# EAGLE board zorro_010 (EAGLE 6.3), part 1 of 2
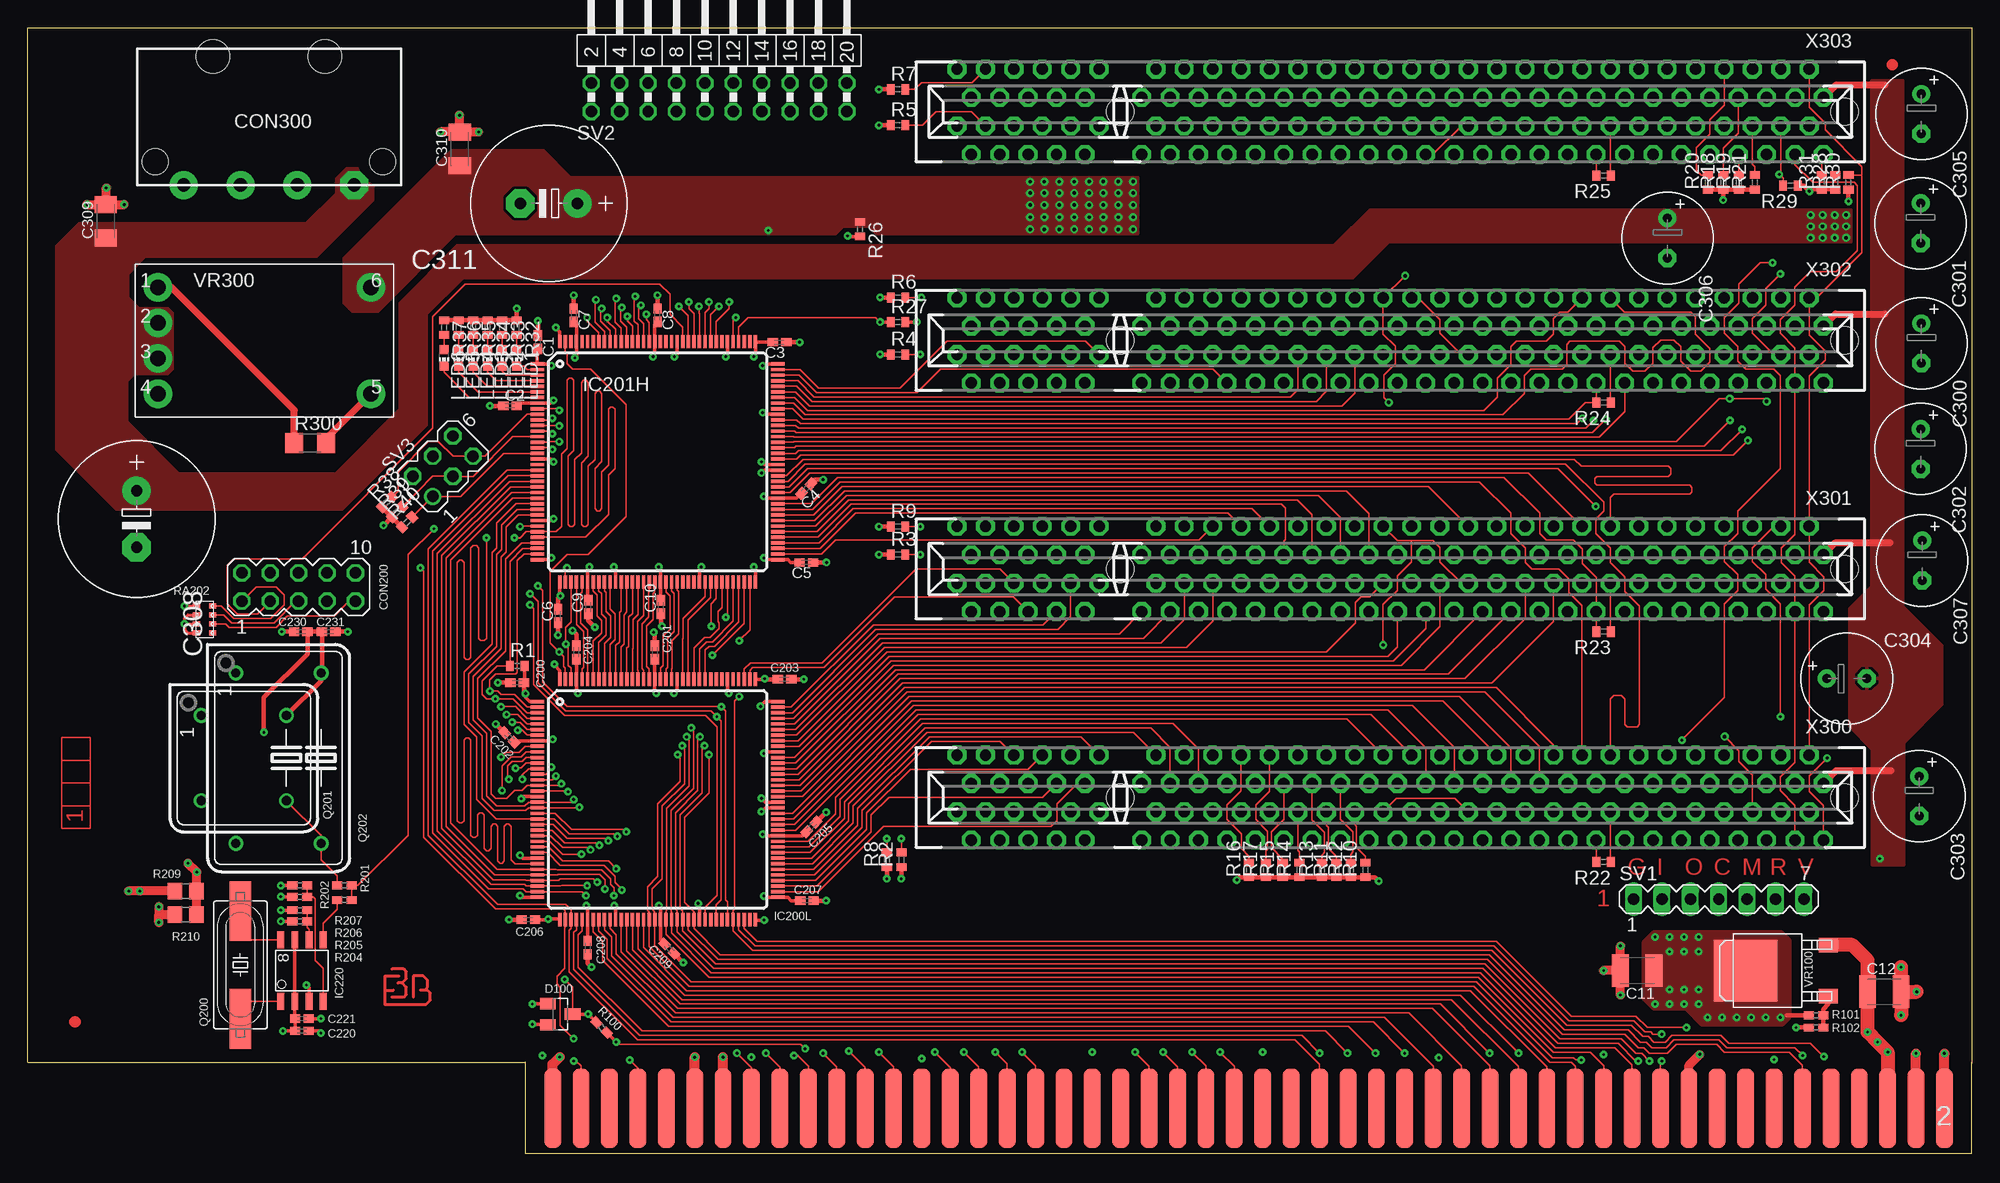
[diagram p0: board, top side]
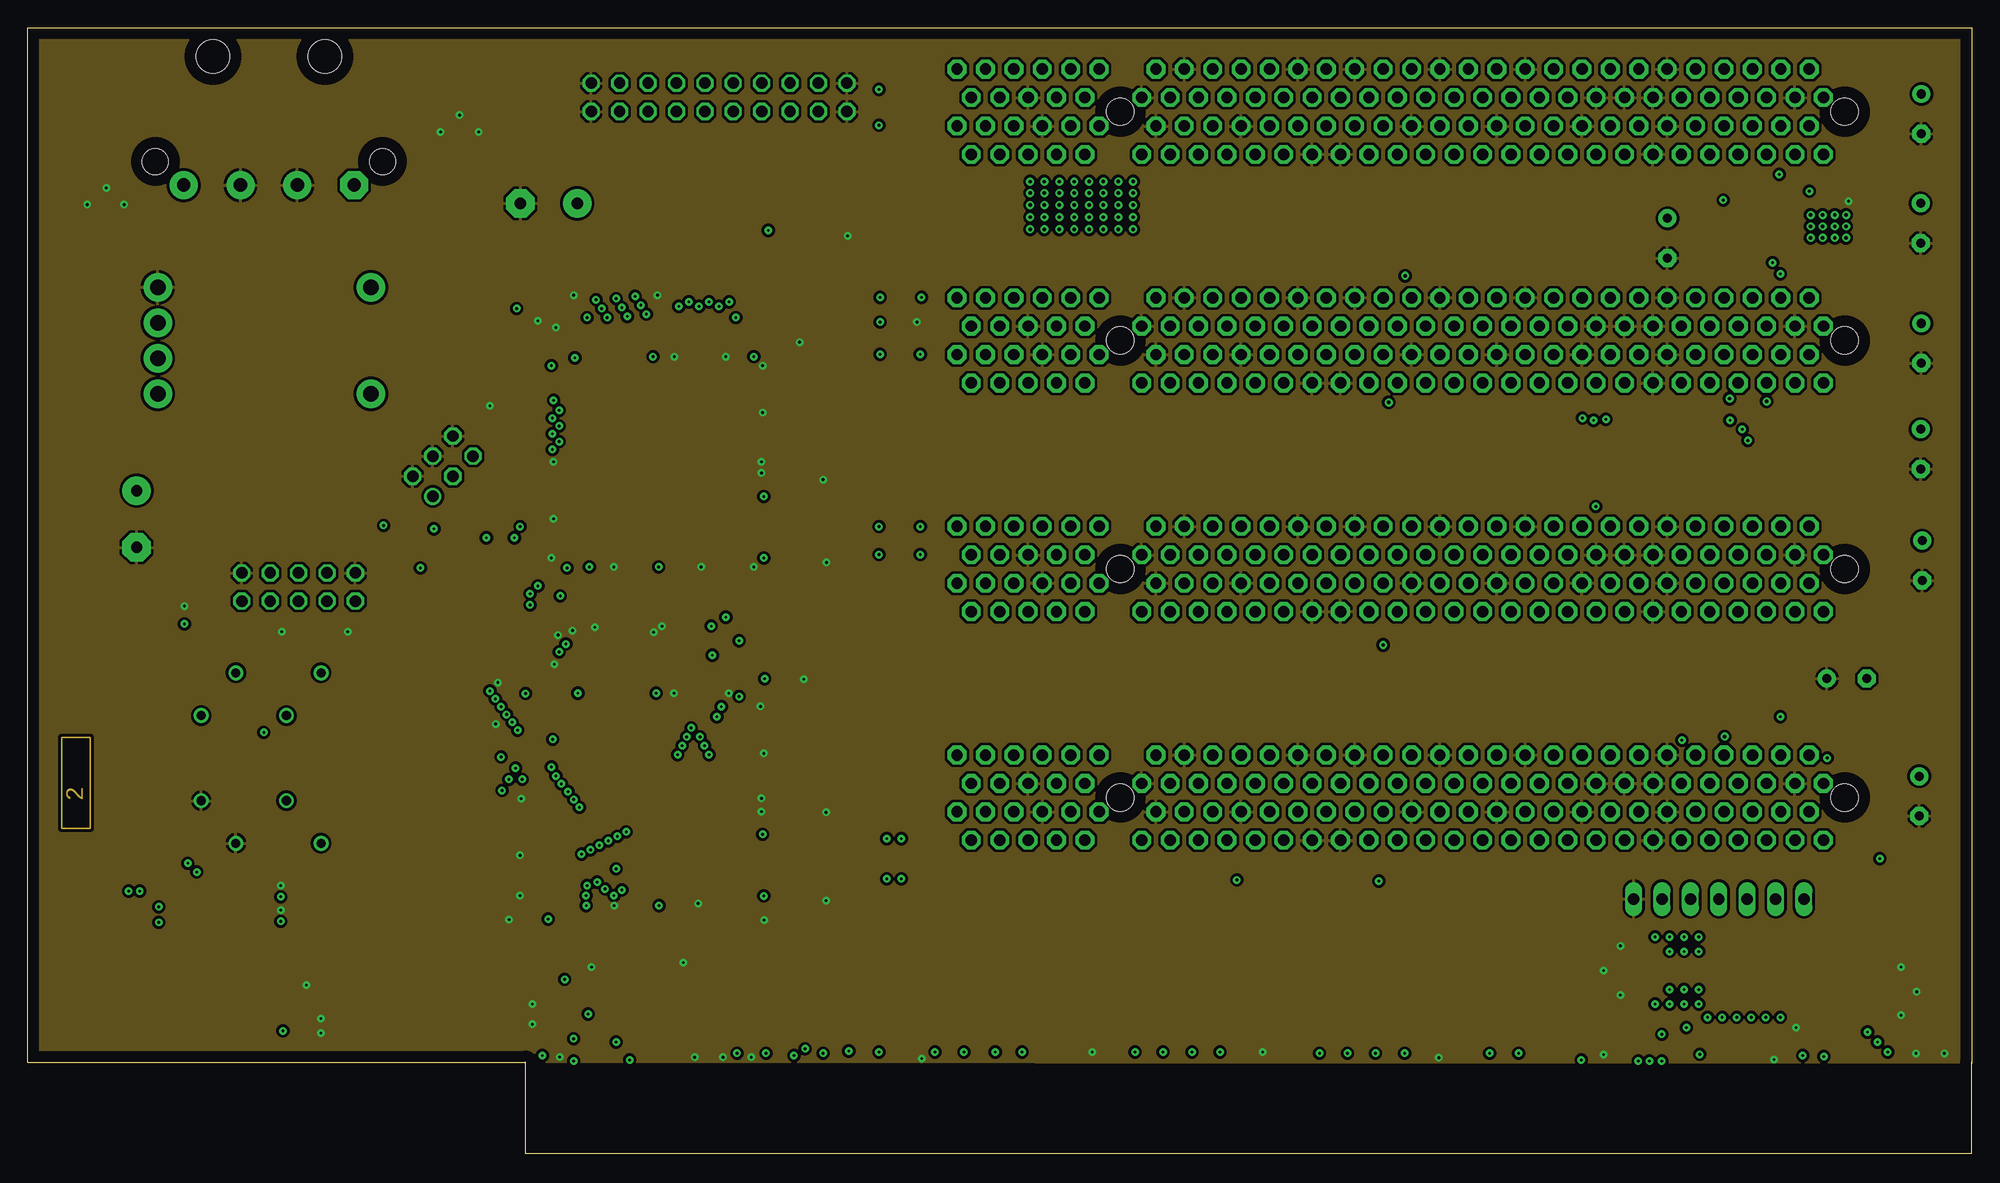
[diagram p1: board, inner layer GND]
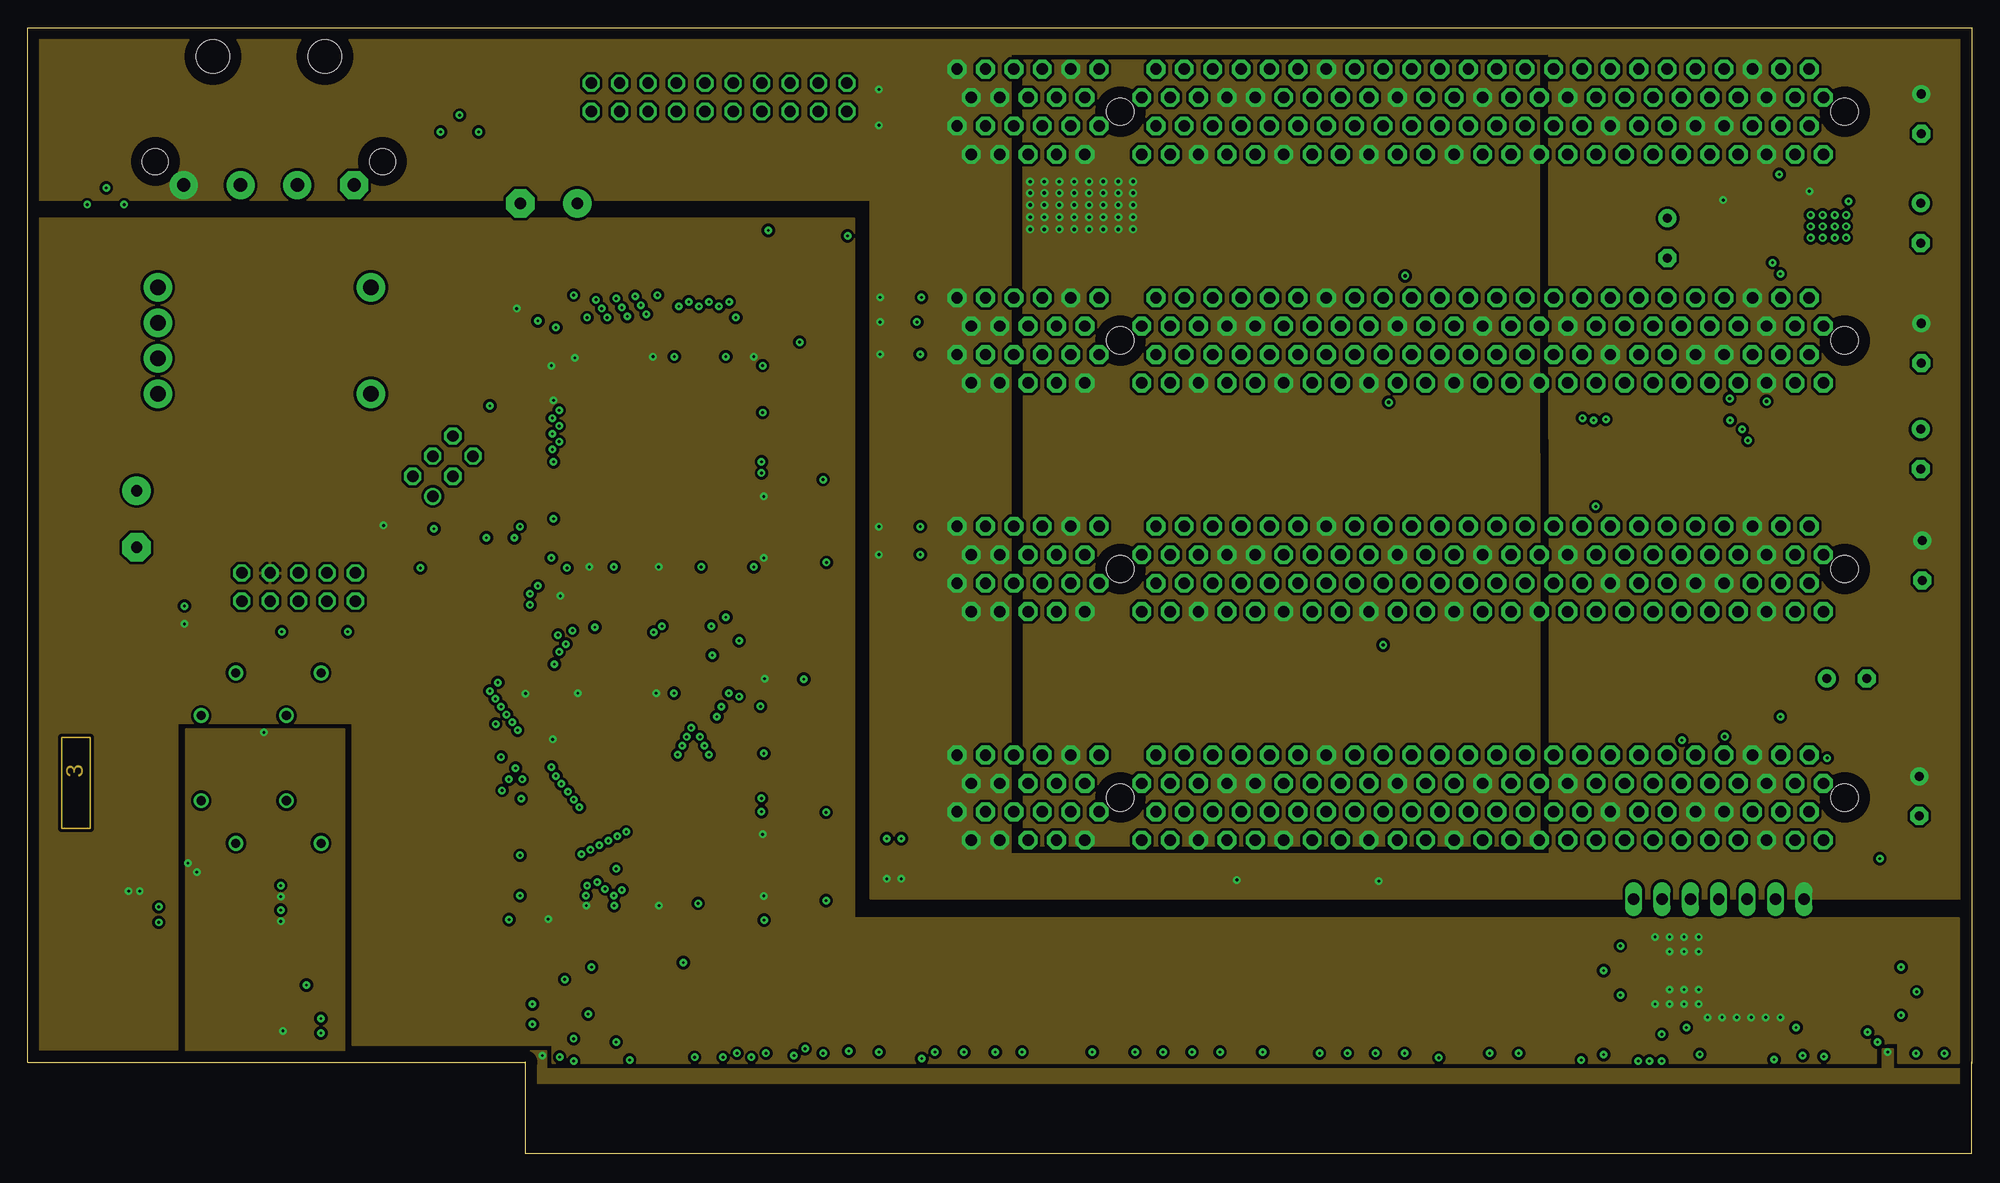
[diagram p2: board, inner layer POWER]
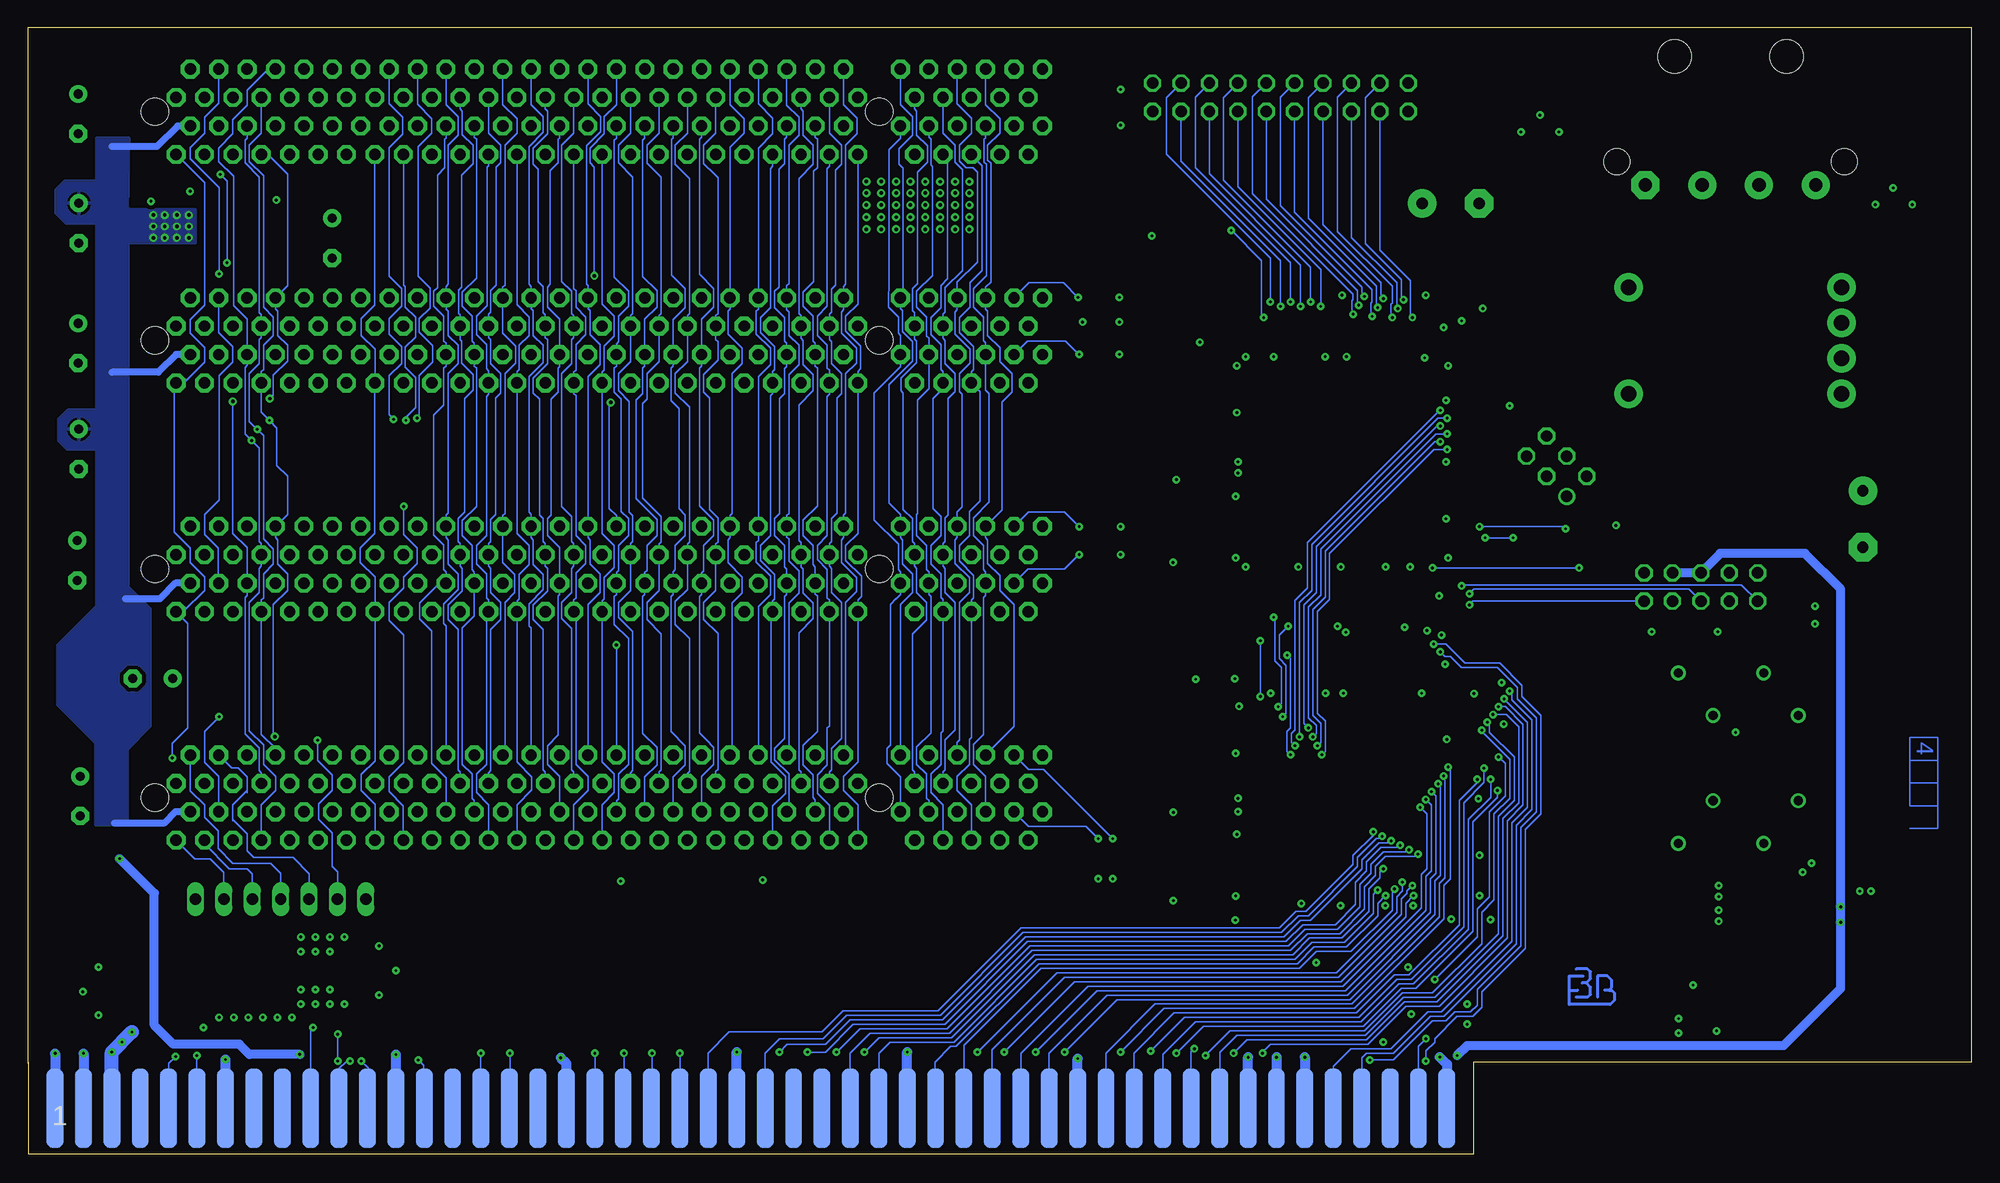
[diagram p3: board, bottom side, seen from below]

Size 173.8 x 100.67 mm. Coordinates in mm from the lower left corner, seen from the top.
Outline: 173.8,8.07 173.8,100.67 0,100.67 0,8.17 44.5,8.17
Copper layers (1+2*15+16): Top 0.035mm / dielectric 0.2mm / GND 0.035mm / dielectric 1.5mm / POWER 0.035mm / dielectric 0.2mm / Bottom 0.035mm
Design rules "default": minimum track width 6mil, minimum drill 8mil, track to track 6mil, track to pad 6mil, pad to pad 6mil, via to via 6mil, smd to smd 6mil, copper to edge 40mil, drill to drill 12mil, minimum pad ring 10mil, minimum via ring 8mil, stop-mask expansion 0mil, vias tented up to drill 0mil, thermal gap 10mil

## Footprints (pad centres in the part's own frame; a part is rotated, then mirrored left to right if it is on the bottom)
C0402K = smd 0.925 x 0.74: 1 -0.6,0; 2 0.6,0
C1210K = smd 1.5 x 2.9: 1 -1.5,0; 2 1.5,0
E3,5-8 = drill 0.813 pad 1.6: + -1.778,0 | drill 0.813 pad 1.6 octagon: - 1.778,0
E5-13 = drill 1.016 pad 2.54: + -2.54,0 | drill 1.016 pad 2.54 octagon: - 2.54,0
C1206K = smd 1.5 x 2: 1 -1.5,0; 2 1.5,0
ZORROM = smd 1.524 x 7.096 bottom: 1 0,4.08; 3 -2.54,4.08; 5 -5.08,4.08; 7 -7.62,4.08; 9 -10.16,4.08; 11 -12.7,4.08; 13 -15.24,4.08; 15 -17.78,4.08; 17 -20.32,4.08; 19 -22.86,4.08; 21 -25.4,4.08; 23 -27.94,4.08; 25 -30.48,4.08; 27 -33.02,4.08; 29 -35.56,4.08; 31 -38.1,4.08; 33 -40.64,4.08; 35 -43.18,4.08; 37 -45.72,4.08; 39 -48.26,4.08; 41 -50.8,4.08; 43 -53.34,4.08; 45 -55.88,4.08; 47 -58.42,4.08; 49 -60.96,4.08; 51 -63.5,4.08; 53 -66.04,4.08; 55 -68.58,4.08; 57 -71.12,4.08; 59 -73.66,4.08; 61 -76.2,4.08; 63 -78.74,4.08; 65 -81.28,4.08; 67 -83.82,4.08; 69 -86.36,4.08; 71 -88.9,4.08; 73 -91.44,4.08; 75 -93.98,4.08; 77 -96.52,4.08; 79 -99.06,4.08; 81 -101.6,4.08; 83 -104.14,4.08; 85 -106.68,4.08; 87 -109.22,4.08; 89 -111.76,4.08; 91 -114.3,4.08; 93 -116.84,4.08; 95 -119.38,4.08; 97 -121.92,4.08; 99 -124.46,4.08 | smd 1.524 x 7.096: 2 0,4.08; 4 -2.54,4.08; 6 -5.08,4.08; 8 -7.62,4.08; 10 -10.16,4.08; 12 -12.7,4.08; 14 -15.24,4.08; 16 -17.78,4.08; 18 -20.32,4.08; 20 -22.86,4.08; 22 -25.4,4.08; 24 -27.94,4.08; 26 -30.48,4.08; 28 -33.02,4.08; 30 -35.56,4.08; 32 -38.1,4.08; 34 -40.64,4.08; 36 -43.18,4.08; 38 -45.72,4.08; 40 -48.26,4.08; 42 -50.8,4.08; 44 -53.34,4.08; 46 -55.88,4.08; 48 -58.42,4.08; 50 -60.96,4.08; 52 -63.5,4.08; 54 -66.04,4.08; 56 -68.58,4.08; 58 -71.12,4.08; 60 -73.66,4.08; 62 -76.2,4.08; 64 -78.74,4.08; 66 -81.28,4.08; 68 -83.82,4.08; 70 -86.36,4.08; 72 -88.9,4.08; 74 -91.44,4.08; 76 -93.98,4.08; 78 -96.52,4.08; 80 -99.06,4.08; 82 -101.6,4.08; 84 -104.14,4.08; 86 -106.68,4.08; 88 -109.22,4.08; 90 -111.76,4.08; 92 -114.3,4.08; 94 -116.84,4.08; 96 -119.38,4.08; 98 -121.92,4.08; 100 -124.46,4.08
MA05-2 = drill 1.016 octagon: 1 -5.08,-1.27; 2 -5.08,1.27; 3 -2.54,-1.27; 4 -2.54,1.27; 5 0,-1.27; 6 0,1.27; 7 2.54,-1.27; 8 2.54,1.27; 9 5.08,-1.27; 10 5.08,1.27
5.25A = drill 1.2 pad 2.5 octagon: 1 -7.62,0 | drill 1.2 pad 2.5: 2 -2.54,0; 3 2.54,0; 4 7.62,0 | hole 2.3: -10.16,-2.1; 10.16,-2.1 | hole 3: -5,-11.5; 5,-11.5
SOT23 = smd 1 x 1.4: 1 -0.95,-1.1; 2 0.95,-1.1; 3 0,1.1
TQFP144 = smd 1.2 x 0.3: 1 -10.75,8.75; 2 -10.75,8.25; 3 -10.75,7.75; 4 -10.75,7.25; 5 -10.75,6.75; 6 -10.75,6.25; 7 -10.75,5.75; 8 -10.75,5.25; 9 -10.75,4.75; 10 -10.75,4.25; 11 -10.75,3.75; 12 -10.75,3.25; 13 -10.75,2.75; 14 -10.75,2.25; 15 -10.75,1.75; 16 -10.75,1.25; 17 -10.75,0.75; 18 -10.75,0.25; 19 -10.75,-0.25; 20 -10.75,-0.75; 21 -10.75,-1.25; 22 -10.75,-1.75; 23 -10.75,-2.25; 24 -10.75,-2.75; 25 -10.75,-3.25; 26 -10.75,-3.75; 27 -10.75,-4.25; 28 -10.75,-4.75; 29 -10.75,-5.25; 30 -10.75,-5.75; 31 -10.75,-6.25; 32 -10.75,-6.75; 33 -10.75,-7.25; 34 -10.75,-7.75; 35 -10.75,-8.25; 36 -10.75,-8.75; 73 10.75,-8.75; 74 10.75,-8.25; 75 10.75,-7.75; 76 10.75,-7.25; 77 10.75,-6.75; 78 10.75,-6.25; 79 10.75,-5.75; 80 10.75,-5.25; 81 10.75,-4.75; 82 10.75,-4.25; 83 10.75,-3.75; 84 10.75,-3.25; 85 10.75,-2.75; 86 10.75,-2.25; 87 10.75,-1.75; 88 10.75,-1.25; 89 10.75,-0.75; 90 10.75,-0.25; 91 10.75,0.25; 92 10.75,0.75; 93 10.75,1.25; 94 10.75,1.75; 95 10.75,2.25; 96 10.75,2.75; 97 10.75,3.25; 98 10.75,3.75; 99 10.75,4.25; 100 10.75,4.75; 101 10.75,5.25; 102 10.75,5.75; 103 10.75,6.25; 104 10.75,6.75; 105 10.75,7.25; 106 10.75,7.75; 107 10.75,8.25; 108 10.75,8.75 | smd 0.3 x 1.2: 37 -8.75,-10.75; 38 -8.25,-10.75; 39 -7.75,-10.75; 40 -7.25,-10.75; 41 -6.75,-10.75; 42 -6.25,-10.75; 43 -5.75,-10.75; 44 -5.25,-10.75; 45 -4.75,-10.75; 46 -4.25,-10.75; 47 -3.75,-10.75; 48 -3.25,-10.75; 49 -2.75,-10.75; 50 -2.25,-10.75; 51 -1.75,-10.75; 52 -1.25,-10.75; 53 -0.75,-10.75; 54 -0.25,-10.75; 55 0.25,-10.75; 56 0.75,-10.75; 57 1.25,-10.75; 58 1.75,-10.75; 59 2.25,-10.75; 60 2.75,-10.75; 61 3.25,-10.75; 62 3.75,-10.75; 63 4.25,-10.75; 64 4.75,-10.75; 65 5.25,-10.75; 66 5.75,-10.75; 67 6.25,-10.75; 68 6.75,-10.75; 69 7.25,-10.75; 70 7.75,-10.75; 71 8.25,-10.75; 72 8.75,-10.75; 109 8.75,10.75; 110 8.25,10.75; 111 7.75,10.75; 112 7.25,10.75; 113 6.75,10.75; 114 6.25,10.75; 115 5.75,10.75; 116 5.25,10.75; 117 4.75,10.75; 118 4.25,10.75; 119 3.75,10.75; 120 3.25,10.75; 121 2.75,10.75; 122 2.25,10.75; 123 1.75,10.75; 124 1.25,10.75; 125 0.75,10.75; 126 0.25,10.75; 127 -0.25,10.75; 128 -0.75,10.75; 129 -1.25,10.75; 130 -1.75,10.75; 131 -2.25,10.75; 132 -2.75,10.75; 133 -3.25,10.75; 134 -3.75,10.75; 135 -4.25,10.75; 136 -4.75,10.75; 137 -5.25,10.75; 138 -5.75,10.75; 139 -6.25,10.75; 140 -6.75,10.75; 141 -7.25,10.75; 142 -7.75,10.75; 143 -8.25,10.75; 144 -8.75,10.75
SO8 = smd 0.61 x 1.524: 1 -1.905,-2.743; 2 -0.635,-2.743; 3 0.635,-2.743; 4 1.905,-2.743; 5 1.905,2.743; 6 0.635,2.743; 7 -0.635,2.743; 8 -1.905,2.743
CHIP-LED0603 = smd 0.8 x 0.8: A 0,-0.75; C 0,0.75
HC49UP = smd 5.334 x 1.93: 1 -4.826,0; 2 4.826,0
DIL08S = drill 0.813: 1 -3.81,-3.81; 4 3.81,-3.81; 5 3.81,3.81; 8 -3.81,3.81
DIL14S = drill 0.813: 1 -7.62,-3.81; 7 7.62,-3.81; 8 7.62,3.81; 14 -7.62,3.81
R0402 = smd 0.7 x 0.9: 1 -0.65,0; 2 0.65,0
R0402@1 = smd 0.9 x 0.7: 1 -0.65,0; 2 0.65,0
R0805@1 = smd 1.3 x 1.5: 1 -0.95,0; 2 0.95,0
R1206 = smd 1.6 x 1.803: 1 -1.422,0; 2 1.422,0
RARRAY4 = smd 0.45 x 0.65: 1 -1.2,-0.725; 2 -0.4,-0.725; 3 0.4,-0.725; 4 1.2,-0.725; 5 1.2,0.725; 6 0.4,0.725; 7 -0.4,0.725; 8 -1.2,0.725
MA07-1 = drill 1.016 long: 1 -7.62,0; 2 -5.08,0; 3 -2.54,0; 4 0,0; 5 2.54,0; 6 5.08,0; 7 7.62,0
MA10-2W = drill 1.016 octagon: 1 -11.43,-1.27; 2 -11.43,1.27; 3 -8.89,-1.27; 4 -8.89,1.27; 5 -6.35,-1.27; 6 -6.35,1.27; 7 -3.81,-1.27; 8 -3.81,1.27; 9 -1.27,-1.27; 10 -1.27,1.27; 11 1.27,-1.27; 12 1.27,1.27; 13 3.81,-1.27; 14 3.81,1.27; 15 6.35,-1.27; 16 6.35,1.27; 17 8.89,-1.27; 18 8.89,1.27; 19 11.43,-1.27; 20 11.43,1.27
MA03-2 = drill 1.016: 1 -2.54,-1.27 | drill 1.016 octagon: 2 -2.54,1.27; 3 0,-1.27; 4 0,1.27; 5 2.54,-1.27; 6 2.54,1.27
TO252 = smd 1.3 x 1.7: 1 -2.285,-7.4; 3 2.285,-7.4 | smd 5.5 x 5.7: 2 0,0
PME_TH = drill 1.397 pad 2.54: 1 -9.525,4.763; 2 -9.525,1.587; 3 -9.525,-1.587; 4 -9.525,-4.763; 5 9.525,-4.763; 6 9.525,4.763
CON-PCI = drill 1.016 pad 1.676 octagon: A1 -38.735,3.81; A2 -37.465,1.27; A3 -36.195,3.81; A4 -34.925,1.27; A5 -33.655,3.81; A6 -32.385,1.27; A7 -31.115,3.81; A8 -29.845,1.27; A9 -28.575,3.81; A10 -27.305,1.27; A11 -26.035,3.81; A12 -24.765,1.27; A13 -23.495,3.81; A14 -22.225,1.27; A15 -20.955,3.81; A16 -19.685,1.27; A17 -18.415,3.81; A18 -17.145,1.27; A19 -15.875,3.81; A20 -14.605,1.27; A21 -13.335,3.81; A22 -12.065,1.27; A23 -10.795,3.81; A24 -9.525,1.27; A25 -8.255,3.81; A26 -6.985,1.27; A27 -5.715,3.81; A28 -4.445,1.27; A29 -3.175,3.81; A30 -1.905,1.27; A31 -0.635,3.81; A32 0.635,1.27; A33 1.905,3.81; A34 3.175,1.27; A35 4.445,3.81; A36 5.715,1.27; A37 6.985,3.81; A38 8.255,1.27; A39 9.525,3.81; A40 10.795,1.27; A41 12.065,3.81; A42 13.335,1.27; A43 14.605,3.81; A44 15.875,1.27; A45 17.145,3.81; A46 18.415,1.27; A47 19.685,3.81; A48 20.955,1.27; A49 22.225,3.81; A52 26.035,1.27; A53 27.305,3.81; A54 28.575,1.27; A55 29.845,3.81; A56 31.115,1.27; A57 32.385,3.81; A58 33.655,1.27; A59 34.925,3.81; A60 36.195,1.27; A61 37.465,3.81; A62 38.735,1.27; B1 -38.735,-1.27; B2 -37.465,-3.81; B3 -36.195,-1.27; B4 -34.925,-3.81; B5 -33.655,-1.27; B6 -32.385,-3.81; B7 -31.115,-1.27; B8 -29.845,-3.81; B9 -28.575,-1.27; B10 -27.305,-3.81; B11 -26.035,-1.27; B12 -24.765,-3.81; B13 -23.495,-1.27; B14 -22.225,-3.81; B15 -20.955,-1.27; B16 -19.685,-3.81; B17 -18.415,-1.27; B18 -17.145,-3.81; B19 -15.875,-1.27; B20 -14.605,-3.81; B21 -13.335,-1.27; B22 -12.065,-3.81; B23 -10.795,-1.27; B24 -9.525,-3.81; B25 -8.255,-1.27; B26 -6.985,-3.81; B27 -5.715,-1.27; B28 -4.445,-3.81; B29 -3.175,-1.27; B30 -1.905,-3.81; B31 -0.635,-1.27; B32 0.635,-3.81; B33 1.905,-1.27; B34 3.175,-3.81; B35 4.445,-1.27; B36 5.715,-3.81; B37 6.985,-1.27; B38 8.255,-3.81; B39 9.525,-1.27; B40 10.795,-3.81; B41 12.065,-1.27; B42 13.335,-3.81; B43 14.605,-1.27; B44 15.875,-3.81; B45 17.145,-1.27; B46 18.415,-3.81; B47 19.685,-1.27; B48 20.955,-3.81; B49 22.225,-1.27; B52 26.035,-3.81; B53 27.305,-1.27; B54 28.575,-3.81; B55 29.845,-1.27; B56 31.115,-3.81; B57 32.385,-1.27; B58 33.655,-3.81; B59 34.925,-1.27; B60 36.195,-3.81; B61 37.465,-1.27; B62 38.735,-3.81 | hole 2.438: 24.13,0; -40.64,0

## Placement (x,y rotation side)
C1  100n  [C0402K]  45.6,72.57 270 top
C2  100n  [C0402K]  43.1,66.87 0 top
C3  100n  [C0402K]  67.2,72.57 180 top
C4  100n  [C0402K]  69.6,59.47 225 top
C5  100n  [C0402K]  69.6,52.87 180 top
C6  100n  [C0402K]  47.4,48.07 90 top
C7  100n  [C0402K]  48.8,74.97 270 top
C8  100n  [C0402K]  56.3,74.97 270 top
C9  100n  [C0402K]  50.1,48.87 90 top
C10  100n  [C0402K]  56.6,48.87 90 top
C11  [C1210K]  143.9,16.37 180 top
C12  [C1210K]  166,14.47 0 top
C200  100n  [C0402K]  43.75,42.12 0 top
C201  100n  [C0402K]  56.05,44.82 270 top
C202  100n  [C0402K]  43.05,37.22 315 top
C203  100n  [C0402K]  67.65,42.42 180 top
C204  100n  [C0402K]  49.05,44.82 270 top
C205  100n  [C0402K]  70.05,29.22 225 top
C206  100n  [C0402K]  44.75,20.92 0 top
C207  100n  [C0402K]  69.65,22.62 180 top
C208  100n  [C0402K]  50.05,18.42 90 top
C209  100n  [C0402K]  57.35,18.32 135 top
C220  DNU  [C0402K]  24.5,10.97 180 top
C221  DNU  [C0402K]  24.5,12.07 180 top
C230  100n  [C0402K]  24.4,46.67 0 top
C231  10n  [C0402K]  26.9,46.67 180 top
C300  [E3,5-8]  169.32,72.48 270 top
C301  [E3,5-8]  169.25,83.21 270 top
C302  [E3,5-8]  169.25,63.02 270 top
C303  [E3,5-8]  169.13,31.96 270 top
C304  [E3,5-8]  162.65,42.48 0 top
C305  [E3,5-8]  169.32,92.99 270 top
C306  [E3,5-8]  146.61,81.87 270 top
C307  [E3,5-8]  169.38,53.05 270 top
C308  [E5-13]  9.72,56.75 270 top
C309  [C1206K]  6.95,83.38 90 top
C310  [C1206K]  38.61,89.84 90 top
C311  [E5-13]  46.58,84.98 180 top
CON100  ZORRO3MEDIUM  [ZORROM]  171.38,-0.03 0 top
CON200  DNU  [MA05-2]  24.2,50.67 0 top
CON300  [5.25A]  21.55,86.62 180 top
D100  BAT54C  [SOT23]  47.6,12.47 270 top
FID100  FIDUCIALJENS  [FID_JENS]  4.2,11.77 0 top
FID101  FIDUCIALJENS  [FID_JENS]  166.7,97.37 0 top
IC200L  XC95144XL  [TQFP144]  56.3,31.67 0 top
IC201H  XC95144XL  [TQFP144]  56.3,61.87 0 top
IC220  DNU  [SO8]  24.5,16.37 0 top
LED1  [CHIP-LED0603]  43.7,71.17 180 top
LED2  [CHIP-LED0603]  42.4,71.17 180 top
LED3  [CHIP-LED0603]  41.1,71.17 180 top
LED4  [CHIP-LED0603]  39.8,71.17 180 top
LED5  [CHIP-LED0603]  38.5,71.17 180 top
LED6  [CHIP-LED0603]  37.2,71.17 180 top
Q200  DNU  [HC49UP]  19,16.87 90 top
Q201  [DIL08S]  19.3,35.37 270 top
Q202  [DIL14S]  22.4,35.37 270 top
R1  DNU  [R0402]  43.75,43.62 0 top
R2  1k0  [R0402]  78.1,26.27 90 top
R3  1k0  [R0402]  77.8,53.57 0 top
R4  1j0  [R0402]  77.8,71.47 0 top
R5  1k0  [R0402]  77.8,91.97 0 top
R6  1j0  [R0402]  77.8,76.57 0 top
R7  1j0  [R0402]  77.8,95.17 0 top
R8  1j0  [R0402]  76.8,26.27 90 top
R9  1j0  [R0402]  77.8,56.07 0 top
R10  1j0  [R0402]  119.6,25.37 90 top
R11  1j0  [R0402]  117,25.37 90 top
R12  1j0  [R0402]  118.3,25.37 90 top
R13  1j0  [R0402]  115.7,25.37 90 top
R14  1j0  [R0402]  113.7,25.37 90 top
R15  1j0  [R0402]  112.2,25.37 90 top
R16  1j0  [R0402]  109.2,25.37 90 top
R17  1j0  [R0402]  110.7,25.37 90 top
R18  1j0  [R0402]  151.6,86.87 90 top
R19  1j0  [R0402]  153,86.87 90 top
R20  1j0  [R0402]  150.2,86.87 90 top
R21  1j0  [R0402]  154.4,86.87 90 top
R22  1j0  [R0402]  140.9,26.07 180 top
R23  1j0  [R0402]  140.9,46.67 180 top
R24  1j0  [R0402]  140.9,67.17 180 top
R25  1j0  [R0402]  140.9,87.47 180 top
R26  3k3  [R0402]  74.4,82.67 270 top
R27  4k7  [R0402]  77.8,74.37 0 top
R28  1j0  [R0402]  161.6,86.87 90 top
R29  1j0  [R0402]  157.6,86.57 180 top
R30  1j0  [R0402]  162.8,86.87 90 top
R31  1j0  [R0402]  160.4,86.87 90 top
R32  3k3  [R0402]  43.7,73.87 270 top
R33  4k7  [R0402]  42.4,73.87 270 top
R34  3k3  [R0402]  41.1,73.87 270 top
R35  4k7  [R0402]  39.8,73.87 270 top
R36  3k3  [R0402]  38.5,73.87 270 top
R37  4k7  [R0402]  37.2,73.87 270 top
R38  4k7  [R0402]  32.1,58.27 45 top
R39  3k3  [R0402]  33,57.37 45 top
R40  4k7  [R0402]  33.9,56.47 45 top
R100  15R0  [R0402@1]  51.3,11.27 135 top
R101  150R0  [R0402@1]  159.9,12.37 180 top
R102  240R0  [R0402@1]  159.9,11.27 0 top
R201  15R0  [R0402@1]  28.3,23.97 0 top
R202  DNU  [R0402@1]  28.3,22.67 0 top
R204  DNU  [R0402@1]  24.3,20.77 180 top
R205  DNU  [R0402@1]  24.3,22.97 180 top
R206  DNU  [R0402@1]  24.3,21.77 0 top
R207  DNU  [R0402@1]  24.3,23.97 0 top
R209  FERRIT  [R0805@1]  14.1,23.47 0 top
R210  FERRIT  [R0805@1]  14.1,21.37 0 top
R300  [R1206]  25.24,63.54 0 top
RA202  DNU  [RARRAY4]  15.8,47.77 270 top
SV1  [MA07-1]  151.2,22.77 0 top
SV2  [MA10-2W]  61.8,94.47 0 top
SV3  [MA03-2]  37.1,61.47 45 top
VR100  GS1117A  [TO252]  153.6,16.37 90 top
VR300  [PME_TH]  21.14,72.71 0 top
X300  [CON-PCI]  121.82,31.84 180 top
X301  [CON-PCI]  121.82,52.28 180 top
X302  [CON-PCI]  121.82,72.73 180 top
X303  [CON-PCI]  121.82,93.18 180 top

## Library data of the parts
C1-C12 C200-C209 C220 C221 C230 C231 C300-C311 R1-R40 R100-R102 R201 R202 R204-R207 R209 R210 R300 = rcl
CON100 CON300 IC200L IC201H IC220 RA202 = AMIGA2
CON200 = con-lstb
D100 = diode
FID100 FID101 VR100 = tum_amiga2
LED1-LED6 = led
Q200-Q202 = crystal
SV1-SV3 = con-lstb; OC_FARNELL: unknown; OC_NEWARK: unknown
VR300 = pola
X300-X303 = con-pc

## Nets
+3V3: C310.1 C311.+ IC201H.113 R26.1 VR300.6 X300.A21 X300.A27 X300.A33 X300.A39 X300.A45 X300.A53 X300.B25 X300.B31 X300.B36 X300.B41 X300.B43 X300.B54 X301.A21 X301.A27 X301.A33 X301.A39 X301.A45 X301.A53 X301.B25 X301.B31 X301.B36 X301.B41 X301.B43 X301.B54 X302.A21 X302.A27 X302.A33 X302.A39 X302.A45 X302.A53 X302.B25 X302.B31 X302.B36 X302.B41 X302.B43 X302.B54 X303.A21 X303.A27 X303.A33 X303.A39 X303.A45 X303.A53 X303.B25 X303.B31 X303.B36 X303.B41 X303.B43 X303.B54
+5V0: C300.+ C303.+ C305.+ C307.+ CON300.4 IC201H.112 R2.1 R3.1 R4.1 R5.1 R6.1 R7.1 R8.1 R9.1 R10.1 R11.1 R12.1 R13.1 R14.1 R15.1 R16.1 R17.1 R18.1 R19.1 R20.1 R21.1 R22.1 R23.1 R24.1 R25.1 R27.1 R28.1 R29.1 R31.1 SV1.7 X300.A5 X300.A8 X300.A10 X300.A16 X300.A59 X300.A61 X300.A62 X300.B5 X300.B6 X300.B19 X300.B59 X300.B61 X300.B62 X301.A5 X301.A8 X301.A10 X301.A16 X301.A59 X301.A61 X301.A62 X301.B5 X301.B6 X301.B19 X301.B59 X301.B61 X301.B62 X302.A5 X302.A8 X302.A10 X302.A16 X302.A59 X302.A61 X302.A62 X302.B5 X302.B6 X302.B19 X302.B59 X302.B61 X302.B62 X303.A5 X303.A8 X303.A10 X303.A16 X303.A59 X303.A61 X303.A62 X303.B5 X303.B6 X303.B19 X303.B59 X303.B61 X303.B62
+12V0: C301.+ C302.+ C306.+ C308.+ C309.1 CON300.1 VR300.2 VR300.3 X300.A2 X301.A2 X302.A2 X303.A2
+12VDC: CON100.10
-12V0: C304.- CON100.20 X300.B1 X301.B1 X302.B1 X303.B1
/BERR: CON100.46 IC200L.39 IC201H.20
/CFGIN: CON100.12 IC200L.60
/CFGOUT: CON100.11 IC200L.61 IC201H.70
/CINH: CON100.17
/DS0: CON100.51 IC200L.22 IC201H.26
/DS1: CON100.98 IC200L.142 IC201H.39
/DS2: CON100.70 IC200L.19 IC201H.28
/DS3: CON100.72 IC200L.16 IC201H.33
/DTACK: CON100.66 IC200L.33 IC201H.23
/FCS: CON100.97 IC200L.38 IC201H.38
/INT2: CON100.19 IC200L.70
/INT6: CON100.22 IC200L.69
/IORST: CON100.94 IC200L.143 IC201H.143
/SLAVE: CON100.9 IC200L.68 IC201H.71
AD8: CON100.30 IC200L.52
AD9: CON100.32 IC200L.50
AD10: CON100.34 IC200L.48
AD11: CON100.36 IC200L.46
AD12: CON100.38 IC200L.45
AD13: CON100.39 IC200L.44
AD14: CON100.41 IC200L.43
AD15: CON100.43 IC200L.41
AD16: CON100.45 IC200L.40
AD17: CON100.47 IC200L.21
AD18: CON100.52 IC200L.23
AD19: CON100.54 IC200L.24
AD20: CON100.56 IC200L.25
AD21: CON100.58 IC200L.27
AD22: CON100.57 IC200L.26
AD23: CON100.59 IC200L.28
AD24: CON100.80 IC200L.10
AD25: CON100.78 IC200L.12
AD26: CON100.76 IC200L.14
AD27: CON100.71 IC200L.17
AD28: CON100.69 IC200L.20 IC201H.27
AD29: CON100.67 IC200L.34 IC201H.22
AD30: CON100.65 IC200L.32 IC201H.24
AD31: CON100.63 IC200L.31 IC201H.25
CLKSEL0: IC220.6 R204.1 R206.2
CLKSEL1: IC220.4 R205.1 R207.2
CLKX1: IC220.1 Q200.1
CLKX2: IC220.8 Q200.2
DEBUG0: IC201H.116 SV2.18
DEBUG1: IC201H.117 SV2.17
DEBUG2: IC201H.118 SV2.16
DEBUG3: IC201H.119 SV2.15
DEBUG4: IC201H.120 SV2.14
DEBUG5: IC201H.121 SV2.13
DEBUG6: IC201H.128 SV2.12
DEBUG7: IC201H.129 SV2.11
DEBUG8: IC201H.130 SV2.10
DEBUG9: IC201H.131 SV2.9
DEBUG10: IC201H.132 SV2.8
DEBUG11: IC201H.133 SV2.7
DEBUG12: IC201H.134 SV2.6
DEBUG13: IC201H.135 SV2.5
DEBUG14: IC201H.136 SV2.4
DEBUG15: IC201H.137 SV2.3
DOE: CON100.93 IC200L.2 IC201H.35
E7M: CON100.92
FC0: CON100.31 IC200L.51
FC1: CON100.33 IC200L.49
FC2: CON100.35
GND: C1.1 C2.1 C3.1 C4.1 C5.1 C6.1 C7.1 C8.1 C9.1 C10.1 C11.2 C12.2 C200.1 C201.1 C202.1 C203.1 C204.1 C205.1 C206.1 C207.1 C208.1 C209.1 C220.1 C221.1 C230.1 C231.1 C300.- C301.- C302.- C303.- C304.+ C305.- C306.- C307.- C308.- C309.2 C310.2 C311.- CON100.1 CON100.2 CON100.3 CON100.4 CON100.13 CON100.25 CON100.37 CON100.49 CON100.61 CON100.73 CON100.85 CON100.87 CON100.88 CON100.89 CON100.90 CON100.99 CON100.100 CON200.2 CON200.10 CON300.2 CON300.3 D100.1 D100.2 IC200L.18 IC200L.29 IC200L.36 IC200L.47 IC200L.62 IC200L.72 IC200L.89 IC200L.90 IC200L.99 IC200L.108 IC200L.114 IC200L.123 IC200L.144 IC201H.18 IC201H.29 IC201H.36 IC201H.47 IC201H.62 IC201H.72 IC201H.89 IC201H.90 IC201H.99 IC201H.108 IC201H.114 IC201H.123 IC201H.144 IC220.3 Q201.4 Q202.7 R26.2 R27.2 R30.1 R102.1 R206.1 R207.1 R300.1 RA202.1 SV1.1 SV2.1 SV2.2 SV2.19 SV2.20 SV3.2 SV3.4 SV3.6 VR300.1 X300.A12 X300.A13 X300.A18 X300.A24 X300.A30 X300.A35 X300.A37 X300.A42 X300.A48 X300.A56 X300.B3 X300.B12 X300.B13 X300.B15 X300.B17 X300.B22 X300.B28 X300.B34 X300.B38 X300.B46 X300.B49 X300.B57 X301.A12 X301.A13 X301.A18 X301.A24 X301.A30 X301.A35 X301.A37 X301.A42 X301.A48 X301.A56 X301.B3 X301.B12 X301.B13 X301.B15 X301.B17 X301.B22 X301.B28 X301.B34 X301.B38 X301.B46 X301.B49 X301.B57 X302.A12 X302.A13 X302.A18 X302.A24 X302.A30 X302.A35 X302.A37 X302.A42 X302.A48 X302.A56 X302.B3 X302.B12 X302.B13 X302.B15 X302.B17 X302.B22 X302.B28 X302.B34 X302.B38 X302.B46 X302.B49 X302.B57 X303.A12 X303.A13 X303.A18 X303.A24 X303.A30 X303.A35 X303.A37 X303.A42 X303.A48 X303.A56 X303.B3 X303.B12 X303.B13 X303.B15 X303.B17 X303.B22 X303.B28 X303.B34 X303.B38 X303.B46 X303.B49 X303.B57
ICON0: IC200L.140 IC201H.40
ICON1: IC200L.139 IC201H.41
ICON2: IC200L.138 IC201H.43
ICON3: IC200L.137 IC201H.44
ICON4: IC200L.136 IC201H.45
ICON5: IC200L.135 IC201H.46
ICON6: IC200L.134 IC201H.48
ICON7: IC200L.133 IC201H.49
ICON8: IC200L.132 IC201H.50
ICON9: IC200L.131 IC201H.51
ICON10: IC200L.130 IC201H.52
ICON11: IC200L.129 IC201H.53
ICON12: IC200L.128 IC201H.54
ICON13: IC200L.126 IC201H.56
ICON14: IC200L.125 IC201H.57
ICON15: IC200L.124 IC201H.58
ICON16: IC200L.121 IC201H.64
ICON17: IC200L.120 IC201H.66
ICON18: IC200L.119 IC201H.68
ICON19: IC200L.118 IC201H.69
LED0: IC201H.2 LED1.C
LED1: IC201H.3 LED2.C
LED2: IC201H.4 LED3.C
LED3: IC201H.5 LED4.C
LED4: IC201H.6 LED5.C
LED5: IC201H.7 LED6.C
MASTERCLK: IC200L.30 IC201H.31 IC201H.32
N$1: R6.2 X302.B60
N$2: R4.2 X302.A60
N$3: R101.1 R102.2 VR100.1
N$6: R5.2 X303.A60
N$9: R7.2 X303.B60
N$10: LED1.A R32.2
N$11: LED2.A R33.2
N$12: LED3.A R34.2
N$13: LED4.A R35.2
N$14: LED5.A R36.2
N$15: LED6.A R37.2
N$18: R2.2 X300.A60
N$19: R300.2 VR300.5
N$21: R3.2 X301.A60
N$22: R9.2 X301.B60
N$40: R8.2 X300.B60
NOTUSED19H: IC201H.19
NOTUSED59H: IC201H.59
NOTUSED60H: IC201H.60
NOTUSED61H: IC201H.61
NOTUSED64L: IC200L.64
NOTUSED66L: IC200L.66
NOTUSED71L: IC200L.71
NOTUSED110H: IC201H.110
NOTUSED111H: IC201H.111
NOTUSED112L: IC200L.112
NOTUSED113L: IC200L.113
NOTUSED115H: IC201H.115
NOTUSED115L: IC200L.115
NOTUSED116L: IC200L.116
NOTUSED117L: IC200L.117
NOTUSED124H: IC201H.124
NOTUSED125H: IC201H.125
NOTUSED126H: IC201H.126
NOTUSED138H: IC201H.138
NOTUSED139H: IC201H.139
NOTUSED140H: IC201H.140
NOTUSED142H: IC201H.142
OPT0: IC201H.10 R38.2 SV3.5
OPT1: IC201H.14 R39.2 SV3.3
OPT2: IC201H.17 R40.2 SV3.1
P-AD0: IC200L.111 X300.A58 X301.A58 X302.A58 X303.A58
P-AD1: IC200L.77 X300.B58 X301.B58 X302.B58 X303.B58
P-AD2: IC200L.110 X300.A57 X301.A57 X302.A57 X303.A57
P-AD3: IC200L.76 X300.B56 X301.B56 X302.B56 X303.B56
P-AD4: IC200L.107 X300.A55 X301.A55 X302.A55 X303.A55
P-AD5: IC200L.75 X300.B55 X301.B55 X302.B55 X303.B55
P-AD6: IC200L.106 X300.A54 X301.A54 X302.A54 X303.A54
P-AD7: IC200L.74 X300.B53 X301.B53 X302.B53 X303.B53
P-AD8: IC200L.78 X300.B52 X301.B52 X302.B52 X303.B52
P-AD9: IC200L.105 X300.A49 X301.A49 X302.A49 X303.A49
P-AD10: IC200L.79 X300.B48 X301.B48 X302.B48 X303.B48
P-AD11: IC200L.104 X300.A47 X301.A47 X302.A47 X303.A47
P-AD12: IC200L.80 X300.B47 X301.B47 X302.B47 X303.B47
P-AD13: IC200L.103 X300.A46 X301.A46 X302.A46 X303.A46
P-AD14: IC200L.81 X300.B45 X301.B45 X302.B45 X303.B45
P-AD15: IC200L.102 X300.A44 X301.A44 X302.A44 X303.A44
P-AD16: IC200L.101 X300.A26 X300.A32 X301.A32 X302.A32 X303.A32
P-AD17: IC200L.82 X300.B32 X301.A26 X301.B32 X302.B32 X303.B32
P-AD18: IC200L.100 X300.A31 X301.A31 X302.A31 X303.A31
P-AD19: IC200L.83 X300.B30 X301.B30 X302.A26 X302.B30 X303.B30
P-AD20: IC200L.98 X300.A29 X301.A29 X302.A29 X303.A26 X303.A29
P-AD21: IC200L.85 X300.B29 X301.B29 X302.B29 X303.B29
P-AD22: IC200L.97 X300.A28 X301.A28 X302.A28 X303.A28
P-AD23: IC200L.86 X300.B27 X301.B27 X302.B27 X303.B27
P-AD24: IC200L.96 X300.A25 X301.A25 X302.A25 X303.A25
P-AD25: IC200L.87 X300.B24 X301.B24 X302.B24 X303.B24
P-AD26: IC200L.95 X300.A23 X301.A23 X302.A23 X303.A23
P-AD27: IC200L.88 X300.B23 X301.B23 X302.B23 X303.B23
P-AD28: IC200L.94 X300.A22 X301.A22 X302.A22 X303.A22
P-AD29: IC200L.91 X300.B21 X301.B21 X302.B21 X303.B21
P-AD30: IC200L.93 X300.A20 X301.A20 X302.A20 X303.A20
P-AD31: IC200L.92 X300.B20 X301.B20 X302.B20 X303.B20
P-CBE0#: IC201H.107 X300.A52 X301.A52 X302.A52 X303.A52
P-CBE1#: IC201H.74 X300.B44 X301.B44 X302.B44 X303.B44
P-CBE2#: IC201H.80 X300.B33 X301.B33 X302.B33 X303.B33
P-CBE3#: IC201H.81 X300.B26 X301.B26 X302.B26 X303.B26
P-CLK0: IC201H.87 X300.B16
P-CLK1: IC201H.88 X301.B16
P-CLK2: IC201H.101 X302.B16
P-CLK3: IC201H.96 X303.B16
P-DEVSEL#: IC201H.78 R13.2 X300.B37 X301.B37 X302.B37 X303.B37
P-FRAME#: IC201H.103 R10.2 X300.A34 X301.A34 X302.A34 X303.A34
P-GNT0#: IC201H.86 R22.2 X300.A17
P-GNT1#: IC201H.83 R23.2 X301.A17
P-GNT2#: IC201H.100 R24.2 X302.A17
P-GNT3#: IC201H.97 R25.2 X303.A17
P-INTA#: IC201H.93 R18.2 X300.A6 X301.B8 X302.A7 X303.B7
P-INTB#: IC201H.94 R19.2 X300.B7 X301.A6 X302.B8 X303.A7
P-INTC#: IC201H.91 R20.2 X300.A7 X301.B7 X302.A6 X303.B8
P-INTD#: IC201H.92 R21.2 X300.B8 X301.A7 X302.B7 X303.A6
P-IRDY#: IC201H.79 R12.2 X300.B35 X301.B35 X302.B35 X303.B35
P-LOCK#: IC201H.77 R15.2 X300.B39 X301.B39 X302.B39 X303.B39
P-PAR: IC201H.106 X300.A43 X301.A43 X302.A43 X303.A43
P-PERR#: IC201H.76 R17.2 X300.B40 X301.B40 X302.B40 X303.B40
P-REQ0#: IC201H.82 X300.B18
P-REQ1#: IC201H.85 X301.B18
P-REQ2#: IC201H.102 X302.B18
P-REQ3#: IC201H.98 X303.B18
P-RST#: IC201H.95 X300.A15 X301.A15 X302.A15 X303.A15
P-SERR#: IC201H.75 R16.2 X300.B42 X301.B42 X302.B42 X303.B42
P-STOP#: IC201H.105 R14.2 X300.A38 X301.A38 X302.A38 X303.A38
P-TCK: R30.2 SV1.4 X300.B2 X301.B2 X302.B2 X303.B2
P-TDI: R29.2 SV1.2 X303.A4
P-TDI1: X302.A4 X303.B4
P-TDI2: X301.A4 X302.B4
P-TDI3: X300.A4 X301.B4
P-TDO: SV1.3 X300.B4
P-TMS: R28.2 SV1.5 X300.A3 X301.A3 X302.A3 X303.A3
P-TRDY#: IC201H.104 R11.2 X300.A36 X301.A36 X302.A36 X303.A36
P-TRST: R31.2 SV1.6 X300.A1 X301.A1 X302.A1 X303.A1
READ: CON100.68 IC200L.35 IC201H.21
SA2: CON100.27 IC200L.54 IC201H.15
SA3: CON100.26 IC200L.56 IC201H.13
SA4: CON100.24 IC200L.57 IC201H.12
SA5: CON100.21 IC200L.59 IC201H.9
SA6: CON100.23 IC200L.58 IC201H.11
SA7: CON100.28 IC200L.53 IC201H.16
SD0: CON100.75 IC200L.15
SD1: CON100.77 IC200L.13
SD2: CON100.79 IC200L.11
SD3: CON100.81 R100.1
SD3X: D100.3 IC200L.9 R100.2
SD4: CON100.83 IC200L.6
SD5: CON100.86 IC200L.4
SD6: CON100.84 IC200L.5
SD7: CON100.82 IC200L.7
SENSEZ3: CON100.91 IC200L.3 IC201H.34 R1.1
SYSCLK: IC201H.30 R201.2 R202.2
SYSCLK_OSC: Q201.5 Q202.8 R201.1
SYSCLK_PLL: IC220.5 R202.1
TCK: CON200.1 IC200L.67 IC201H.67 RA202.8
TDI: CON200.9 IC200L.63 RA202.6
TDO: CON200.3 IC201H.122
TDO-TDI: IC200L.122 IC201H.63
TMS: CON200.5 IC200L.65 IC201H.65 RA202.7
VCC: C12.1 CON100.5 CON100.6 CON200.6 CON200.8 R210.1 VR100.3
VDD: C1.2 C2.2 C3.2 C4.2 C5.2 C6.2 C7.2 C8.2 C9.2 C10.2 C11.1 C200.2 C201.2 C202.2 C203.2 C204.2 C205.2 C206.2 C207.2 C208.2 C209.2 CON200.4 IC200L.1 IC200L.8 IC200L.37 IC200L.42 IC200L.55 IC200L.73 IC200L.84 IC200L.109 IC200L.127 IC200L.141 IC201H.1 IC201H.8 IC201H.37 IC201H.42 IC201H.55 IC201H.73 IC201H.84 IC201H.109 IC201H.127 IC201H.141 R1.2 R32.1 R33.1 R34.1 R35.1 R36.1 R37.1 R38.1 R39.1 R40.1 R101.2 R209.1 RA202.2 RA202.3 RA202.4 VR100.2
VPP: C220.2 C221.2 C230.2 C231.2 IC220.2 IC220.7 Q201.8 Q202.14 R204.2 R205.2 R209.2 R210.2

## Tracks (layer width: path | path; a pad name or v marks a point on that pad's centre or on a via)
+3V3  (via drill 0.25 pad 0.67, 0.3 pad 0.61)
  Top 0.152: IC201H.113 63.05,74.52 v63.3,74.77
  Bottom 0.152: v63.3,74.77 63.5,74.97 63.5,79.87 v66.2,82.57
  other vias: 93.56,85.91 90.89,85.91 89.62,85.91 92.23,85.91 89.62,84.83 90.89,84.83 92.23,84.83 93.56,84.83 89.62,83.75 90.89,83.75 92.23,83.75 93.56,83.75 93.56,86.93 90.89,86.93 89.62,86.93 92.23,86.93 93.56,82.67 90.89,82.67 89.62,82.67 92.23,82.67 94.89,86.94 96.16,86.94 97.5,86.94 94.89,82.67 94.89,85.91 96.16,85.91 97.5,85.91 96.16,82.67 94.89,84.83 96.16,84.83 97.5,84.83 97.5,82.67 94.89,83.75 96.16,83.75 97.5,83.75 98.83,86.94 98.83,85.91 98.83,84.83 98.83,82.67 98.83,83.75
  pour POWER (isolate 0.254, no thermals): 88.98,97.77 89.04,47.14 89.04,27.52 135.21,27.52 135.14,97.77
  pour Top (isolate 0.254, no thermals): 99.3,87.37 99.3,82.17 75.9,82.17 75.2,82.87 72.9,82.87 72.2,82.17 38.2,82.17 31.3,75.27 29,75.27 28.2,76.07 28.2,80.07 37.9,89.77 46.1,89.77 48.5,87.37
+5V0  (via drill 0.25 pad 0.67)
  Top 0.152: X301.A16 141.5,46.72 R23.1 | X300.A16 141.5,26.12 R22.1 | X302.A16 141.5,67.22 R24.1 | X303.A16 141.5,87.52 R25.1 | IC201H.112 63.55,73.92 64.4,74.77 75.8,74.77 v76.2,74.37
  Top 0.305: v76.2,74.37 R27.1 | R28.1 R31.1 159.45,86.22 v159.3,86.07
  Top 0.406: R3.1 v76.1,53.57 | R9.1 v76.1,56.07 | R6.1 v76.2,76.57 | R4.1 v76.2,71.47 | R7.1 v76.1,95.17 | R5.1 v76.1,91.97 | v76.8,24.57 R8.1 | v78.1,24.57 R2.1 | R29.1 158.8,86.57 v159.3,86.07 | R21.1 R19.1 R18.1 | R18.1 v151.6,85.27 | R20.1 R18.1 | v120.8,24.37 120.45,24.72 R10.1 R12.1 R11.1 R13.1 R14.1 R15.1 R17.1 R16.1 108.35,24.72 v108.1,24.47
  pour POWER (isolate 0.254, no thermals): 0,100.97 135.9,100.97 135.88,98.33 87.9,98.33 87.9,26.82 136.03,26.82 136,100.97 178.5,100.97 178.5,22.77 75.3,22.77 75.3,85.27 0,85.27
+12V0  (via drill 0.3 pad 0.61)
  Bottom 0.61: X303.A2 160.43,91.91 162.27,90.07 166.27,90.07 | X302.A2 160.55,71.46 162.14,69.87 166.27,69.87 | X301.A2 160.62,51.01 162.01,49.62 165.06,49.62 | X300.A2 160.62,30.57 161.63,29.55 166.08,29.55
  other vias: 162.59,83.94 161.57,83.94 160.49,83.94 159.41,83.94 159.41,82.93 160.49,82.93 161.57,82.93 162.59,82.93 162.59,81.91 161.57,81.91 160.49,81.91 159.41,81.91
  pour Bottom (isolate 0.356): 164.94,29.42 164.94,36.16 162.9,38.19 162.9,48.73 164.87,50.7 164.87,81.47 158.87,81.47 158.87,84.4 164.91,84.4 164.81,90.83 167.67,90.83 167.67,86.96 170.52,86.96 171.28,86.19 171.28,84.1 170.4,83.21 167.67,83.21 167.67,66.51 170.21,66.51 171.03,65.68 171.03,63.78 170.27,63.02 167.67,63.02 167.67,48.92 171.16,45.43 171.16,40.16 167.73,36.73 167.73,29.42
  pour Top (isolate 0.254, no thermals): 163.1,84.47 163.1,81.47 121.7,81.47 118.5,78.27 38.9,78.27 35.7,75.07 35.7,65.17 28.1,57.57 27.5,57.57 7.9,57.57 2.5,62.97 2.5,81.17 4.6,83.27 24.9,83.27 27.5,85.87 27.5,87.17 28.5,88.17 29.8,88.17 30.9,87.07 30.9,85.27 25.8,80.17 10.5,80.17 9,78.67 9,76.57 9.9,75.67 12.5,75.67 13,75.17 13,70.17 12.5,69.67 9.5,69.67 8.9,69.07 8.9,65.47 13.5,60.87 27.5,60.87 33.2,66.57 33.2,76.07 38.4,81.27 116.8,81.27 120,84.47
-12V0  (via drill 0.25 pad 0.67)
  Top 0.61: X303.B1 161.7,95.59 166.08,95.59 | X302.B1 161.63,75.08 166.08,75.08 | X301.B1 161.63,54.63 166.52,54.63 | X300.B1 161.7,34.25 166.59,34.25
  Top 0.813: CON100.20 148.52,7.89 v149.5,8.87
  Bottom 0.813: v149.5,8.87 154,8.87 154.9,9.77 160.8,9.77 162.5,11.47 162.5,23.27 v165.6,26.37
  pour Top (isolate 0.356): 167.67,48.92 167.67,95.97 164.87,95.97 164.87,50.7 162.9,48.73 162.9,38.19 164.94,36.16 164.94,25.81 167.73,25.81 167.73,36.73 171.16,40.16 171.16,45.43
/BERR
  Top 0.152: CON100.46 115.5,7.97 113.3,10.17 54.5,10.17 48.4,16.27 48.4,19.97 48.55,20.12 IC200L.39 48.55,21.82 48.1,22.27 42,22.27 35.8,28.47 35.8,29.77 35.8,54.07 42.85,61.12 IC201H.20
/CFGIN
  Top 0.152: CON100.12 158.68,7.89 157.5,9.07 151.7,9.07 151,9.77 147.4,9.77 146.6,8.97 145,8.97 144.5,9.47 144,9.47 142.8,10.67 137.2,10.67 130.5,17.37 61.7,17.37 59.05,20.02 IC200L.60
/CFGOUT  (via drill 0.25 pad 0.67)
  Top 0.152: v158.7,8.77 158,9.47 151.9,9.47 151.2,10.17 147.2,10.17 146.5,9.47 145.2,9.47 144.7,9.97 144.2,9.97 143.1,11.07 137.4,11.07 130.7,17.77 61.9,17.77 59.55,20.12 IC200L.61 59.55,21.62 58.7,22.47 58.7,30.07 60.9,32.27 v60.9,35.67 | IC201H.70 64.05,47.42 v61.2,44.57
  Bottom 0.152: CON100.11 158.7,4.07 v158.7,8.77 | v60.9,35.67 61.2,35.97 61.2,37.77 60.9,38.07 60.9,44.27 v61.2,44.57
/DS0  (via drill 0.25 pad 0.67)
  Top 0.152: v52.7,28.37 52.5,28.57 48.4,28.57 47.05,29.92 IC200L.22 41.85,29.92 40.1,31.67 40.1,37.27 39,38.37 39,43.07 41.5,45.57 41.5,53.77 41.9,54.17 41.9,56.37 43.65,58.12 IC201H.26
  Bottom 0.152: CON100.51 107.9,4.07 107.9,8.97 106.6,10.27 102.7,10.27 100.6,12.37 92.2,12.37 84.8,19.77 61.7,19.77 60.2,21.27 59.3,21.27 54.9,25.67 54.9,26.47 53.2,28.17 52.9,28.17 v52.7,28.37
/DS1  (via drill 0.25 pad 0.67)
  Top 0.152: CON100.98 49.46,7.83 49.02,8.27 v48.8,8.27 | IC200L.142 48.55,43.42 48.3,43.67 48.3,45.37 v48.1,45.57 48.1,47.07 48.55,47.52 IC201H.39
  Bottom 0.152: v48.1,45.57 47,45.57 45.3,43.87 42.2,43.87 40.2,41.87 40.2,40.87 38.5,39.17 38.5,30.37 39.9,28.97 39.9,18.37 43.8,14.47 43.8,13.07 44.6,12.27 46,12.27 48,10.27 48,9.97 48.8,9.17 v48.8,8.27
/DS2  (via drill 0.25 pad 0.67)
  Top 0.152: CON100.70 85.02,7.75 v83.7,9.07 | v48.8,31.67 48.55,31.42 IC200L.19 44.75,31.42 44.4,31.07 41.9,31.07 41,31.97 41,37.57 39.8,38.77 39.8,42.67 42.3,45.17 42.3,53.37 42.75,53.82 42.75,56.02 43.85,57.12 IC201H.28
  Bottom 0.152: v48.8,31.67 48.3,31.17 48.3,25.27 48.8,24.77 48.8,21.77 56,14.57 78.2,14.57 v83.7,9.07
/DS3  (via drill 0.25 pad 0.67)
  Top 0.152: CON100.72 82.48,7.69 v81.1,9.07 | v47.7,33.07 47.55,32.92 IC200L.16 44.65,32.92 44.2,32.47 43.5,32.47 42.8,31.77 41.8,31.77 41.4,32.17 41.4,37.77 40.2,38.97 40.2,42.47 42.7,44.97 42.7,53.17 44.15,54.62 IC201H.33
  Bottom 0.152: v47.7,33.07 47.5,32.87 47.5,24.87 48,24.37 48,21.37 55.6,13.77 76.4,13.77 v81.1,9.07
/DTACK  (via drill 0.25 pad 0.67)
  Top 0.152: CON100.66 90.1,7.87 v88.9,9.07 | v50.9,24.27 50.6,24.57 47.6,24.57 47.45,24.42 IC200L.33 44.55,24.42 44.5,24.47 41.6,24.47 37,29.07 37,30.37 37,53.47 43.15,59.62 IC201H.23
  Bottom 0.152: v50.9,24.27 50.9,23.47 51.4,22.97 51.4,21.57 56.8,16.17 81.8,16.17 v88.9,9.07
/FCS  (via drill 0.25 pad 0.66, 0.25 pad 0.67)
  Top 0.152: v48.8,10.27 47.6,11.47 47.6,14.87 47.3,15.17 47.3,15.87 48,16.57 48,20.17 48.05,20.22 IC200L.38 48.05,21.72 47.9,21.87 41.8,21.87 35.4,28.27 35.4,29.57 35.4,52.07 v35.1,52.37 | IC201H.38 48.05,52.22 v48.2,52.37
  Bottom 0.152: CON100.97 49.46,9.61 v48.8,10.27 | v35.1,52.37 v48.2,52.37
/INT2  (via drill 0.25 pad 0.67)
  Top 0.152: v148.3,11.27 144.8,11.27 143.8,12.27 138,12.27 131.3,18.97 65.2,18.97 64.05,20.12 IC200L.70
  Bottom 0.152: CON100.19 148.52,11.05 v148.3,11.27
/INT6  (via drill 0.25 pad 0.67)
  Top 0.152: CON100.22 145.98,8.15 v146.1,8.27 | v146.1,10.67 145.3,10.67 145.1,10.87 144.6,10.87 143.6,11.87 137.8,11.87 131.1,18.57 65,18.57 63.55,20.02 IC200L.69
  Bottom 0.152: v146.1,10.67 v146.1,8.27
/IORST  (via drill 0.25 pad 0.67)
  Top 0.152: CON100.94 54.54,7.63 v53.8,8.37 | IC200L.143 48.05,43.42 47.9,43.57 47.9,44.47 v47.5,44.87 46.7,45.67 46.7,52.07 48.2,53.57 50.1,53.57 53.5,56.97 53.5,66.97 50.3,70.17 48.7,70.17 48.2,70.67 48.2,71.57 48.05,71.72 IC201H.143
  Bottom 0.152: v47.5,44.87 47.1,44.47 46.6,44.47 45.6,43.47 42.4,43.47 40.6,41.67 40.6,40.67 38.9,38.97 38.9,30.57 40.3,29.17 40.3,18.57 44.2,14.67 44.2,13.27 44.8,12.67 46.2,12.67 47,11.87 48.2,11.87 51.7,8.37 v53.8,8.37
/SLAVE  (via drill 0.25 pad 0.67)
  Top 0.152: v160.6,8.67 159.4,9.87 152.1,9.87 151.4,10.57 147,10.57 146.4,9.97 145.4,9.97 144.9,10.47 144.4,10.47 143.4,11.47 137.6,11.47 130.9,18.17 64.8,18.17 63.05,19.92 IC200L.68 63.05,21.72 63.2,21.87 63.2,40.47 v63.6,40.87 | IC201H.71 64.55,46.82 v63.6,45.87
  Bottom 0.152: CON100.9 161.2,4.07 161.2,8.07 v160.6,8.67 | v63.6,40.87 v63.6,45.87
AD8
  Top 0.152: CON100.30 135.82,7.75 129,14.57 58.9,14.57 55.05,18.42 IC200L.52
AD9
  Top 0.152: CON100.32 133.28,7.79 127.3,13.77 58.5,13.77 54.05,18.22 IC200L.50
AD10
  Top 0.152: CON100.34 130.74,7.83 125.6,12.97 58.1,12.97 53.05,18.02 IC200L.48
AD11
  Top 0.152: CON100.36 128.2,7.87 123.5,12.57 57.9,12.57 52.6,17.87 52.6,19.57 52.05,20.12 IC200L.46
AD12
  Top 0.152: CON100.38 125.66,7.81 121.3,12.17 57.7,12.17 52.2,17.67 52.2,19.37 51.55,20.02 IC200L.45
AD13  (via drill 0.25 pad 0.67)
  Top 0.152: v123.1,8.97 120.3,11.77 57.5,11.77 51.8,17.47 51.8,19.17 51.05,19.92 IC200L.44
  Bottom 0.152: CON100.39 123.1,4.07 v123.1,8.97
AD14  (via drill 0.25 pad 0.67)
  Top 0.152: v120.5,8.97 118.1,11.37 57.3,11.37 51.4,17.27 51.4,18.97 50.55,19.82 IC200L.43
  Bottom 0.152: CON100.41 120.5,4.13 v120.5,8.97
AD15  (via drill 0.25 pad 0.67)
  Top 0.152: v118,8.97 116,10.97 54.9,10.97 49.2,16.67 49.2,19.57 49.55,19.92 IC200L.41
  Bottom 0.152: CON100.43 118,4.09 v118,8.97
AD16  (via drill 0.25 pad 0.67)
  Top 0.152: v115.5,8.97 113.9,10.57 54.7,10.57 48.8,16.47 48.8,19.77 49.05,20.02 IC200L.40
  Bottom 0.152: CON100.45 v115.5,8.97
AD17  (via drill 0.25 pad 0.67)
  Top 0.152: IC200L.21 47.15,30.42 48.6,28.97 53.3,28.97 v53.5,28.77
  Bottom 0.152: CON100.47 113,4.09 113,8.97 111.1,10.87 102.8,10.87 100.9,12.77 92.4,12.77 85,20.17 61.9,20.17 60.4,21.67 59.5,21.67 55.3,25.87 55.3,26.67 53.5,28.47 v53.5,28.77
AD18  (via drill 0.25 pad 0.67)
  Top 0.152: CON100.52 107.88,7.79 v106.6,9.07 | IC200L.23 46.95,29.42 48.2,28.17 51.7,28.17 v51.9,27.97
  Bottom 0.152: v106.6,9.07 105.9,9.77 102.5,9.77 100.3,11.97 92,11.97 84.6,19.37 61.5,19.37 60,20.87 59.1,20.87 54.5,25.47 54.5,26.27 53,27.77 52.1,27.77 v51.9,27.97
AD19  (via drill 0.25 pad 0.67)
  Top 0.152: CON100.54 105.34,7.83 v104.1,9.07 | IC200L.24 46.85,28.92 48,27.77 50.9,27.77 v51.1,27.57
  Bottom 0.152: v104.1,9.07 102.5,9.07 100,11.57 91.8,11.57 84.4,18.97 61.3,18.97 59.8,20.47 56.9,20.47 55.1,22.27 55.1,24.27 54.1,25.27 54.1,26.07 52.8,27.37 51.3,27.37 v51.1,27.57
AD20  (via drill 0.25 pad 0.67)
  Top 0.152: CON100.56 102.8,7.77 v101.5,9.07 | IC200L.25 46.75,28.42 47.8,27.37 50.1,27.37 v50.3,27.17
  Bottom 0.152: v101.5,9.07 99.4,11.17 91.6,11.17 84.2,18.57 61.1,18.57 59.6,20.07 56.7,20.07 54.7,22.07 54.7,24.07 53.7,25.07 53.7,25.87 52.6,26.97 50.5,26.97 v50.3,27.17
AD21  (via drill 0.25 pad 0.67)
  Top 0.152: CON100.58 100.26,7.81 v99,9.07 | IC200L.27 46.55,27.42 47.8,26.17 51.9,26.17 v52.6,25.47
  Bottom 0.152: v99,9.07 97.7,10.37 91.2,10.37 83.8,17.77 60.7,17.77 59.2,19.27 56.3,19.27 53.9,21.67 53.9,23.67 52.9,24.67 52.9,25.17 v52.6,25.47
AD22  (via drill 0.25 pad 0.67)
  Top 0.152: IC200L.26 46.65,27.92 47.8,26.77 v49.5,26.77
  Bottom 0.152: CON100.57 100.3,4.09 100.3,8.97 98.5,10.77 91.4,10.77 84,18.17 60.9,18.17 59.4,19.67 56.5,19.67 54.3,21.87 54.3,23.87 53.3,24.87 53.3,25.67 52.4,26.57 49.7,26.57 v49.5,26.77
AD23  (via drill 0.25 pad 0.67)
  Top 0.152: IC200L.28 46.45,26.92 47.6,25.77 51.5,25.77 52.5,24.77 52.5,24.27 53.1,23.67 v53.1,23.57
  Bottom 0.152: CON100.59 97.7,4.07 97.7,8.97 96.7,9.97 91,9.97 83.6,17.37 60.5,17.37 59,18.87 56.1,18.87 53.5,21.47 53.5,23.17 v53.1,23.57
AD24  (via drill 0.25 pad 0.67)
  Top 0.152: CON100.80 72.32,7.75 v71.1,8.97 | IC200L.10 44.55,35.92 44.1,35.47 43.2,35.47 42.4,34.67 v42.4,32.47
  Bottom 0.152: v42.4,32.47 42.4,31.87 44.6,29.67 44.6,19.87 49.7,14.77 51,14.77 54.4,11.37 68.7,11.37 v71.1,8.97
AD25  (via drill 0.25 pad 0.67)
  Top 0.152: CON100.78 74.86,7.71 v73.4,9.17 | IC200L.12 44.55,34.92 44.1,34.47 v43.6,34.47
  Bottom 0.152: v43.6,34.47 43.6,33.17 45.4,31.37 45.4,20.27 50.1,15.57 51.4,15.57 54.8,12.17 70.4,12.17 v73.4,9.17
AD26  (via drill 0.25 pad 0.67)
  Top 0.152: CON100.76 77.4,7.77 v76.1,9.07 | IC200L.14 46.35,33.92 46.6,34.17 46.6,34.37 v46.8,34.57
  Bottom 0.152: v46.8,34.57 46.6,34.37 46.6,24.57 47.2,23.97 47.2,20.97 55.2,12.97 72.2,12.97 v76.1,9.07
AD27  (via drill 0.25 pad 0.67)
  Top 0.152: IC200L.17 48.25,32.42 v48.3,32.37
  Bottom 0.152: CON100.71 82.5,4.07 82.5,8.97 77.3,14.17 55.8,14.17 48.4,21.57 48.4,24.57 47.9,25.07 47.9,31.97 v48.3,32.37
AD28  (via drill 0.25 pad 0.67)
  Top 0.152: v49.3,30.97 49.25,30.92 IC200L.20 44.75,30.92 44.5,30.67 41.7,30.67 40.6,31.77 40.6,37.37 39.4,38.57 39.4,42.87 41.9,45.37 41.9,53.57 42.35,54.02 42.35,56.22 43.75,57.62 IC201H.27
  Bottom 0.152: CON100.69 85,4.07 85,8.97 79,14.97 56.2,14.97 49.2,21.97 49.2,24.97 48.7,25.47 48.7,30.37 v49.3,30.97
AD29  (via drill 0.25 pad 0.67)
  Top 0.152: v50,23.97 47.7,23.97 47.65,23.92 IC200L.34 44.55,23.92 44.4,24.07 41.4,24.07 36.6,28.87 36.6,30.17 36.6,53.67 43.05,60.12 IC201H.22
  Bottom 0.152: CON100.67 87.6,4.09 87.6,9.27 81.1,15.77 56.6,15.77 51,21.37 51,22.77 50.5,23.27 50.5,23.47 v50,23.97
AD30  (via drill 0.25 pad 0.67)
  Top 0.152: v51.6,23.67 51.6,24.47 51.1,24.97 47.4,24.97 47.35,24.92 IC200L.32 41.75,24.92 37.4,29.27 37.4,30.57 37.4,53.27 43.25,59.12 IC201H.24
  Bottom 0.152: CON100.65 90.1,9.67 83.2,16.57 60.1,16.57 58.6,18.07 55.5,18.07 51.8,21.77 51.8,23.47 v51.6,23.67
AD31  (via drill 0.25 pad 0.67)
  Top 0.152: v52.4,23.07 52.4,23.77 52.1,24.07 52.1,24.57 51.3,25.37 47.3,25.37 47.25,25.42 IC200L.31 41.95,25.42 37.8,29.57 37.8,30.77 37.8,53.07 43.35,58.62 IC201H.25
  Bottom 0.152: CON100.63 92.7,4.11 92.7,8.17 91.3,9.57 90.8,9.57 83.4,16.97 60.3,16.97 58.8,18.47 55.9,18.47 53.1,21.27 53.1,22.37 v52.4,23.07
CLKSEL0
  Top 0.152: R206.2 24.95,20.82 25,20.77 R204.1 24.95,20.22 25.14,20.04 IC220.6
CLKSEL1
  Top 0.152: R207.2 24.95,23.02 25,22.97 R205.1 25.5,22.97 25.7,22.77 25.7,17.27 26.41,16.57 IC220.4
CLKX1
  Top 0.152: IC220.1 19,13.63 Q200.1
CLKX2
  Top 0.152: IC220.8 19.56,19.12 19,19.67 Q200.2
DEBUG0  (via drill 0.25 pad 0.67)
  Top 0.152: IC201H.116 61.55,74.42 62.7,75.57 v62.7,76.17
  Bottom 0.152: SV2.18 72,94.43 72,89.37 62.7,80.07 v62.7,76.17
DEBUG1  (via drill 0.25 pad 0.67)
  Top 0.152: IC201H.117 61.05,75.02 v61.8,75.77
  Bottom 0.152: v61.8,75.77 61.8,79.87 70.69,88.76 SV2.17 70.69,93.06
DEBUG2  (via drill 0.25 pad 0.67)
  Top 0.152: IC201H.118 60.55,75.22 60.9,75.57 v60.9,76.17
  Bottom 0.152: SV2.16 69.4,94.49 69.4,88.17 60.9,79.67 v60.9,76.17
DEBUG3  (via drill 0.25 pad 0.67)
  Top 0.152: IC201H.119 60.05,75.12 60,75.17 v60,75.77
  Bottom 0.152: v60,75.77 60,79.47 68.15,87.62 SV2.15
DEBUG4  (via drill 0.25 pad 0.67)
  Top 0.152: IC201H.120 59.55,75.12 59.1,75.57 v59.1,76.17
  Bottom 0.152: SV2.14 66.9,94.45 66.9,87.07 59.1,79.27 v59.1,76.17
DEBUG5  (via drill 0.25 pad 0.67)
  Top 0.152: IC201H.121 59.05,74.92 v58.2,75.77
  Bottom 0.152: v58.2,75.77 58.2,79.07 65.61,86.48 SV2.13
DEBUG6  (via drill 0.25 pad 0.67)
  Top 0.152: IC201H.128 55.55,74.32 55.3,74.57 v55.3,75.07
  Bottom 0.152: v55.3,75.07 55.4,75.17 55.4,76.27 55.3,76.37 55.3,76.87 64.3,85.87 64.3,94.51 SV2.12
DEBUG7  (via drill 0.25 pad 0.67)
  Top 0.152: IC201H.129 55.05,74.22 54.6,74.67 54.6,75.67 v54.8,75.87
  Bottom 0.152: v54.8,75.87 54.9,75.97 54.9,77.17 63.07,85.34 SV2.11
DEBUG8  (via drill 0.25 pad 0.67)
  Top 0.152: IC201H.130 54.55,74.12 54.2,74.47 54.2,76.57 v54.3,76.67
  Bottom 0.152: v54.3,76.67 54.5,76.87 54.5,77.47 61.8,84.77 61.8,94.47 SV2.10
DEBUG9  (via drill 0.25 pad 0.67)
  Top 0.152: IC201H.131 54.05,74.02 53.6,74.47 v53.6,74.87
  Bottom 0.152: v53.6,74.87 53.7,74.97 53.7,76.07 53.6,76.17 53.6,77.27 60.53,84.2 SV2.9
DEBUG10  (via drill 0.25 pad 0.67)
  Top 0.152: IC201H.132 53.55,73.92 53,74.47 53,75.57 v53.1,75.67
  Bottom 0.152: v53.1,75.67 53.2,75.77 53.2,77.57 59.3,83.67 59.3,94.43 SV2.8
DEBUG11  (via drill 0.25 pad 0.67)
  Top 0.152: IC201H.133 53.05,73.82 52.5,74.37 52.5,76.37 v52.6,76.47
  Bottom 0.152: v52.6,76.47 52.8,76.67 52.8,77.87 57.99,83.06 SV2.7
DEBUG12  (via drill 0.25 pad 0.67)
  Top 0.152: IC201H.134 52.55,73.72 51.8,74.47 v51.8,74.77
  Bottom 0.152: v51.8,74.77 51.9,74.87 51.9,75.97 51.8,76.07 51.8,77.57 56.7,82.47 56.7,94.49 SV2.6
DEBUG13  (via drill 0.25 pad 0.67)
  Top 0.152: IC201H.135 52.05,73.62 51.2,74.47 51.2,75.47 v51.3,75.57
  Bottom 0.152: v51.3,75.57 51.4,75.67 51.4,77.87 55.45,81.92 SV2.5
DEBUG14  (via drill 0.25 pad 0.67)
  Top 0.152: IC201H.136 51.55,73.52 50.7,74.37 50.7,76.27 v50.8,76.37
  Bottom 0.152: v50.8,76.37 51,76.57 51,78.17 54.2,81.37 54.2,94.45 SV2.4
DEBUG15  (via drill 0.25 pad 0.67)
  Top 0.152: IC201H.137 51.05,73.42 50,74.47 v50,74.77
  Bottom 0.152: v50,74.77 50.2,74.97 50.2,78.07 52.91,80.78 SV2.3
DOE  (via drill 0.25 pad 0.67)
  Top 0.152: IC200L.2 44.65,39.92 43.5,41.07 42.3,41.07 42,41.37 v41.3,41.37 41.3,42.37 41.8,42.87 43.6,42.87 43.75,43.02 43.75,53.02 44.35,53.62 IC201H.35
  Bottom 0.152: CON100.93 54.5,4.09 54.5,8.57 54.1,8.97 51.7,8.97 48.4,12.27 47.2,12.27 40.7,18.77 40.7,29.37 39.3,30.77 39.3,38.77 41.1,40.57 41.1,41.17 v41.3,41.37
FC0  (via drill 0.25 pad 0.67)
  Top 0.152: v133.3,8.97 128.1,14.17 58.7,14.17 54.55,18.32 IC200L.51
  Bottom 0.152: CON100.31 133.3,4.07 v133.3,8.97
FC1  (via drill 0.25 pad 0.67)
  Top 0.152: v130.7,8.97 126.3,13.37 58.3,13.37 53.55,18.12 IC200L.49
  Bottom 0.152: CON100.33 130.7,4.09 v130.7,8.97
GND  (via drill 0.25 pad 0.67)
  Top 0.254: v14,48.97 RA202.1
  Top 0.305: IC200L.114 62.55,41.3 v62.67,41.17 | IC200L.18 44.27,31.92 v44.1,31.75 | IC200L.108 65.92,40.42 v65.5,40 | IC200L.99 65.92,35.92 v65.8,35.8 | IC200L.90 65.95,31.42 v65.6,31.77 | IC200L.89 65.95,30.92 v65.6,30.57 | IC200L.47 52.55,22.05 v52.42,22.17 | IC200L.62 60.05,22.25 v59.92,22.37 | IC220.3 25.14,14.84 v24.9,15.07 | C221.1 v26.2,12.07 | C220.1 26,10.97 v26.2,10.77 | IC200L.72 65.1,20.87 v65.83,20.87 | IC200L.29 44.25,26.42 v44,26.67 | IC200L.36 44.15,22.92 v44,23.07 | R206.1 v22.6,21.77 | R207.1 v22.6,23.97 | v57.77,41.17 57.8,41.17 58.05,41.42 IC200L.123 | v47.08,43.77 47.08,43.7 47.55,43.22 IC200L.144 | D100.2 46.5,11.57 v45.1,11.57 | D100.1 46.5,13.37 v45.1,13.37 | IC201H.47 52.55,52.32 v52.4,52.47 | IC201H.62 60.05,52.32 v60.2,52.47 | IC201H.36 46.65,53.12 v46.8,53.27 | IC201H.29 46.85,56.62 v47,56.77 | IC201H.18 46.75,62.12 v47,61.87 | IC201H.144 47.55,73.52 v47.2,73.87 | IC201H.114 62.55,71.42 v62.4,71.27 | IC201H.108 65.85,70.62 v65.7,70.47 | IC201H.99 65.85,66.12 v65.7,66.27 | IC201H.90 65.85,61.62 v65.6,61.87 | IC201H.89 65.85,61.12 v65.6,60.87 | IC201H.72 65.05,52.32 v64.9,52.47 | C205.1 70.5,29.65 | IC201H.123 58.05,71.52 v57.8,71.27 | R27.2 v79.5,74.37 | R26.2 73.35,82.02 v73.3,82.07
  Top 0.406: C200.1 v42.02,42.12 | C207.1 v71.38,22.62 | C206.1 v43.02,20.92 | C203.1 v69.38,42.42 | C208.1 50.05,17.02 v50.4,16.67 | v158.1,11.27 R102.1 | v58.6,17.07 C209.1 | C231.1 v28.6,46.67 | C230.1 v22.7,46.67 | C6.1 v47.4,46.37 | v50.7,47.07 50.1,47.67 C9.1 | C201.1 56.05,46.52 v55.95,46.62 | C10.1 56.6,47.27 v56.7,47.17 | v41.3,66.87 C2.1 | C7.1 v48.8,76.77 | C8.1 v56.3,76.77 | C5.1 v71.4,52.87 | C3.1 v69,72.57 | 70.5,29.65 v71.38,30.52 | v71.1,60.27 70.4,60.27 C4.1 | C1.1 v45.6,74.47 | v162.8,85.17 R30.1 | C204.1 49.05,46.42 v48.7,46.77 | C202.1 42.6,37.65 v41.83,38.42
  Top 0.61: R300.1 23.81,66.48 12.82,77.47 VR300.1
  Top 0.813: C310.2 38.6,91.37 | 38.6,91.37 v38.6,92.87 | 38.6,91.37 v36.9,91.37 | 38.6,91.37 v40.3,91.37 | 7,84.88 C309.2 | 7,84.88 v7,86.37 | 7,84.87 7,84.88 | v5.3,84.87 7,84.87 | 7,84.87 v8.6,84.87 | C11.2 v142.4,18.57 | v142.4,14.17 C11.2 | C11.2 v140.9,16.37
  Top 0.914: CON100.4 v168.83,8.96 | CON100.2 v171.37,8.96 | CON100.90 v59.61,8.61 | CON100.88 v62.15,8.61 | CON100.100 46.91,8 v47.55,8.63
  Top 1.27: C12.2 v167.5,16.67 | C12.2 v167.5,12.37 | C12.2 v168.9,14.47
  Bottom 0.914: v126.16,8.58 125.65,8.07 CON100.37 | CON100.2 v171.37,8.96 | CON100.4 v168.83,8.96 | CON100.13 v156.13,8.4 | CON100.25 v140.89,8.86 | CON100.49 v110.41,9.09 | CON100.61 v95.17,9.09 | CON100.73 v79.93,8.49 | CON100.85 v64.69,8.61 | CON100.88 v62.15,8.61 | CON100.90 v59.61,8.61 | CON100.100 46.91,8 v47.55,8.63
  pour GND (isolate 0.254): 0,103.77 0,8.17 180.1,8.07 180.1,103.77
ICON0
  Top 0.152: IC201H.40 49.05,47.32 49.7,46.67 49.7,43.47 49.55,43.32 IC200L.140
ICON1
  Top 0.152: IC201H.41 49.55,50.22 49.4,50.07 49.4,47.47 50.05,46.82 IC200L.139
ICON2
  Top 0.152: IC201H.43 50.55,50.32 50.9,49.97 50.9,48.07 51.3,47.67 51.3,46.57 50.55,45.82 IC200L.138
ICON3
  Top 0.152: IC200L.137 51.05,45.72 51.7,46.37 51.7,47.87 51.3,48.27 51.3,50.07 51.05,50.32 IC201H.44
ICON4
  Top 0.152: IC201H.45 51.55,50.32 51.7,50.17 51.7,48.47 52.1,48.07 52.1,46.17 51.55,45.62 IC200L.136
ICON5
  Top 0.152: IC201H.46 52.05,48.72 52.5,48.27 52.5,45.97 52.05,45.52 IC200L.135
ICON6
  Top 0.152: IC200L.134 52.55,45.42 52.9,45.77 52.9,48.37 53.05,48.52 IC201H.48
ICON7
  Top 0.152: IC201H.49 53.55,48.42 53.3,48.17 53.3,45.57 53.05,45.32 IC200L.133
ICON8
  Top 0.152: IC201H.50 54.05,48.32 53.7,47.97 53.7,45.37 53.55,45.22 IC200L.132
ICON9
  Top 0.152: IC201H.51 54.55,48.22 54.1,47.77 54.1,45.17 54.05,45.12 IC200L.131
ICON10
  Top 0.152: IC201H.52 55.05,48.12 54.5,47.57 54.5,43.27 54.55,43.22 IC200L.130
ICON11
  Top 0.152: IC201H.53 55.55,50.22 55.5,50.17 55.5,47.97 54.9,47.37 54.9,43.37 55.05,43.22 IC200L.129
ICON12
  Top 0.152: IC201H.54 56.05,50.22 55.9,50.07 55.9,47.77 55.3,47.17 55.3,43.57 55.55,43.32 IC200L.128
ICON13
  Top 0.152: IC200L.126 56.55,43.42 56.8,43.67 56.8,46.27 57.4,46.87 57.4,49.87 57.05,50.22 IC201H.56
ICON14
  Top 0.152: IC201H.57 57.55,50.32 57.8,50.07 57.8,46.67 57.2,46.07 57.2,43.47 57.05,43.32 IC200L.125
ICON15
  Top 0.152: IC201H.58 58.05,50.42 58.2,50.27 58.2,46.47 57.6,45.87 57.6,43.37 57.55,43.32 IC200L.124
ICON16
  Top 0.152: IC201H.64 61.05,49.72 59.05,47.72 IC200L.121
ICON17
  Top 0.152: IC201H.66 62.05,48.82 61.7,48.47 61.7,47.57 61.8,47.47 61.8,46.97 61,46.17 60.5,46.17 59.55,45.22 IC200L.120
ICON18
  Top 0.152: IC201H.68 63.05,47.62 61.2,45.77 60.7,45.77 60.05,45.12 IC200L.119
ICON19
  Top 0.152: IC201H.69 63.55,47.52 61.4,45.37 60.9,45.37 60.55,45.02 IC200L.118
LED0
  Top 0.152: IC201H.2 44.65,70.12 44.35,70.42 LED1.C
LED1
  Top 0.152: IC201H.3 42.75,69.62 42.4,69.97 LED2.C
LED2
  Top 0.152: LED3.C 41.1,69.87 41.85,69.12 IC201H.4
LED3
  Top 0.152: LED4.C 39.8,69.87 41.05,68.62 IC201H.5
LED4
  Top 0.152: LED5.C 38.5,69.87 40.25,68.12 IC201H.6
LED5
  Top 0.152: LED6.C 37.2,69.87 39.45,67.62 IC201H.7
MASTERCLK  (via drill 0.25 pad 0.67)
  Top 0.152: IC200L.30 43.55,25.92 43.2,26.27 43.2,29.27 43,29.47 42.8,29.47 42.6,29.27 42.6,26.17 42.4,25.97 42.2,25.97 42,26.17 42,29.27 41.8,29.47 41.6,29.47 41.4,29.27 41.4,27.27 41.2,27.07 41,27.07 40.8,27.27 40.8,30.27 40.6,30.47 40.4,30.47 40.2,30.27 40.2,28.47 40,28.27 39.8,28.27 39.6,28.47 39.6,36.97 39.4,37.17 39.2,37.17 39,36.97 39,29.77 38.8,29.57 38.6,29.57 38.4,29.77 38.4,52.87 38.6,53.07 38.8,53.07 39,52.87 39,44.37 39.2,44.17 39.4,44.17 39.6,44.37 39.6,54.17 39.8,54.37 40.1,54.37 40.3,54.17 40.3,46.07 40.5,45.87 40.8,45.87 41,46.07 v41,55.07 | v43.5,55.07 44,55.07 44.55,55.62 IC201H.31 47.25,55.62 47.7,56.07 47.7,62.57 48.2,63.07 48.2,69.17 48.4,69.37 48.6,69.37 48.8,69.17 48.8,62.87 48.3,62.37 48.3,56.27 48.5,56.07 48.7,56.07 48.9,56.27 48.9,62.07 49.5,62.67 49.5,68.97 49.7,69.17 49.9,69.17 50.1,68.97 50.1,62.37 49.5,61.77 49.5,56.27 49.7,56.07 49.9,56.07 50.1,56.27 50.1,61.47 50.7,62.07 50.7,67.97 50.9,68.17 51.1,68.17 51.3,67.97 51.3,61.87 50.7,61.27 50.7,57.67 50.9,57.47 51.1,57.47 51.3,57.67 51.3,60.97 51.9,61.57 51.9,66.57 52.1,66.77 52.3,66.77 52.5,66.57 52.5,61.27 51.9,60.67 51.9,57.17 49.85,55.12 IC201H.32
  Bottom 0.152: v41,55.07 v43.5,55.07
N$1  (via drill 0.25 pad 0.67)
  Top 0.152: R6.2 v79.9,76.57
  Bottom 0.152: X302.B60 84.29,77.87 81.2,77.87 v79.9,76.57
N$2  (via drill 0.25 pad 0.67)
  Top 0.152: R4.2 v79.8,71.47
  Bottom 0.152: X302.A60 84.41,72.67 81,72.67 v79.8,71.47
N$3
  Top 0.406: VR100.1 161,13.37 160.55,12.92 R101.1 160.55,11.32 160.5,11.27 R102.2
N$4
  Bottom 0.254: 35.99,14.62 35.99,15.89 34.72,15.89 | 35.99,14.62 35.99,13.35 32.3,13.35 31.92,13.73 31.92,14.36 32.18,14.62 32.43,14.62 | 35.99,14.62 35.22,14.62 | 32.43,14.62 32.18,14.87 32.18,15.5 32.56,15.89 33.45,15.89 33.45,13.98 | 32.43,14.62 32.81,14.62
N$6
  Top 0.152: X303.A60 84.36,93.17 81.2,93.17 80,91.97 R5.2
N$7
  Top 0.254: 31.92,14.62 31.92,15.89 33.19,15.89 | 31.92,14.62 31.92,13.35 35.61,13.35 35.99,13.73 35.99,14.36 35.73,14.62 35.48,14.62 | 31.92,14.62 32.68,14.62 | 35.48,14.62 35.73,14.87 35.73,15.5 35.35,15.89 34.46,15.89 34.46,13.98 | 35.48,14.62 35.1,14.62
N$8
